(* Logix 5000 AddOnInstructionDefinition export BMC_AOI_PROC_BNI00HM; software revision 20.04 *)

TYPE BMC_UDT_PROC_BNI00HM_Outputs_4277US :   // BNI EIP-508-005-Z015-013Output Map
STRUCT
   Data : INT;
   Restart : INT;
END_STRUCT
END_TYPE

TYPE BMC_UDT_PROC_BNI00HM_Config_4277US :   // BNI EIP-508-005-Z015-013Configuration Map
STRUCT
   Port_1_Function : SINT;   // Sets Port 1 Function 00d=0x00=Standrd I/O 01d=0x01=IO-Link Mod 02d=0x02=Fallback Md
   Port_2_Function : SINT;   // Sets Port 2 Function 00d=0x00=Standrd I/O 01d=0x01=IO-Link Mod 02d=0x02=Fallback Md
   Port_3_Function : SINT;   // Sets Port 3 Function 00d=0x00=Standrd I/O 01d=0x01=IO-Link Mod 02d=0x02=Fallback Md
   Port_4_Function : SINT;   // Sets Port 4 Function 00d=0x00=Standrd I/O 01d=0x01=IO-Link Mod 02d=0x02=Fallback Md
   Port_5_Function : SINT;   // Sets Port 5 Function 00d=0x00=Standrd I/O 01d=0x01=IO-Link Mod 02d=0x02=Fallback Md
   Port_6_Function : SINT;   // Sets Port 6 Function 00d=0x00=Standrd I/O 01d=0x01=IO-Link Mod 02d=0x02=Fallback Md
   Port_7_Function : SINT;   // Sets Port 7 Function 00d=0x00=Standrd I/O 01d=0x01=IO-Link Mod 02d=0x02=Fallback Md
   Port_8_Function : SINT;   // Sets Port 8 Function 00d=0x00=Standrd I/O 01d=0x01=IO-Link Mod 02d=0x02=Fallback Md
   Port_1_Cycle_Time : SINT;   // This SINT is a composite value. Bits 0-5 store Cycle Time Bit 6-7 store Time Base
   Port_1_Validation_Type : SINT;   // Port 1 Validation 00d=0x00=No Validtn 01d=0x01=Compatible [VID + DID]
   Port_1_Vendor_ID_1 : SINT;   // Vendor ID (Hi Byte) of device connected to Port 1 Balluff VID = 378
   Port_1_Vendor_ID_2 : SINT;   // Vendor ID (Lo Byte)
   Port_1_Device_ID_1 : SINT;   // Device ID (Hi Byte) of device connected to Port 1
   Port_1_Device_ID_2 : SINT;   // Device ID (Mid Byte)
   Port_1_Device_ID_3 : SINT;   // Device ID (Low Byte)
   Enable_Upload_Port_1 : BOOL;
   Enable_Download_Port_1 : BOOL;
   Clear_Parameter_Server_Port_1 : BOOL;
   Enable_Parameter_Server_Port_1 : BOOL;
   Port_2_Cycle_Time : SINT;   // This SINT is a composite value. Bits 0-5 store Cycle Time Bit 6-7 store Time Base
   Port_2_Validation_Type : SINT;   // Port 2 Validation 00d=0x00=No Validtn 01d=0x01=Compatible [VID + DID]
   Port_2_Vendor_ID_1 : SINT;   // Vendor ID (Hi Byte) of device connected to Port 2 Balluff VID = 378
   Port_2_Vendor_ID_2 : SINT;   // Vendor ID (Lo Byte)
   Port_2_Device_ID_1 : SINT;   // Device ID (Hi Byte) of device connected to Port 2
   Port_2_Device_ID_2 : SINT;   // Device ID (Mid Byte)
   Port_2_Device_ID_3 : SINT;   // Device ID (Low Byte)
   Enable_Upload_Port_2 : BOOL;
   Enable_Download_Port_2 : BOOL;
   Clear_Parameter_Server_Port_2 : BOOL;
   Enable_Parameter_Server_Port_2 : BOOL;
   Port_3_Cycle_Time : SINT;   // This SINT is a composite value. Bits 0-5 store Cycle Time Bit 6-7 store Time Base
   Port_3_Validation_Type : SINT;   // Port 3 Validation 00d=0x00=No Validtn 01d=0x01=Compatible [VID + DID]
   Port_3_Vendor_ID_1 : SINT;   // Vendor ID (Hi Byte) of device connected to Port 3 Balluff VID = 378
   Port_3_Vendor_ID_2 : SINT;   // Vendor ID (Lo Byte)
   Port_3_Device_ID_1 : SINT;   // Device ID (Hi Byte) of device connected to Port 3
   Port_3_Device_ID_2 : SINT;   // Device ID (Mid Byte)
   Port_3_Device_ID_3 : SINT;   // Device ID (Low Byte)
   Enable_Upload_Port_3 : BOOL;
   Enable_Download_Port_3 : BOOL;
   Clear_Parameter_Server_Port_3 : BOOL;
   Enable_Parameter_Server_Port_3 : BOOL;
   Port_4_Cycle_Time : SINT;   // This SINT is a composite value. Bits 0-5 store Cycle Time Bit 6-7 store Time Base
   Port_4_Validation_Type : SINT;   // Port 4 Validation 00d=0x00=No Validtn 01d=0x01=Compatible [VID + DID]
   Port_4_Vendor_ID_1 : SINT;   // Vendor ID (Hi Byte) of device connected to Port 4 Balluff VID = 378
   Port_4_Vendor_ID_2 : SINT;   // Vendor ID (Lo Byte)
   Port_4_Device_ID_1 : SINT;   // Device ID (Hi Byte) of device connected to Port 4
   Port_4_Device_ID_2 : SINT;   // Device ID (Mid Byte)
   Port_4_Device_ID_3 : SINT;   // Device ID (Low Byte)
   Enable_Upload_Port_4 : BOOL;
   Enable_Download_Port_4 : BOOL;
   Clear_Parameter_Server_Port_4 : BOOL;
   Enable_Parameter_Server_Port_4 : BOOL;
   Port_5_Cycle_Time : SINT;   // This SINT is a composite value. Bits 0-5 store Cycle Time Bit 6-7 store Time Base
   Port_5_Validation_Type : SINT;   // Port 5 Validation 00d=0x00=No Validtn 01d=0x01=Compatible [VID + DID]
   Port_5_Vendor_ID_1 : SINT;   // Vendor ID (Hi Byte) of device connected to Port 5 Balluff VID = 378
   Port_5_Vendor_ID_2 : SINT;   // Vendor ID (Lo Byte)
   Port_5_Device_ID_1 : SINT;   // Device ID (Hi Byte) of device connected to Port 5
   Port_5_Device_ID_2 : SINT;   // Device ID (Mid Byte)
   Port_5_Device_ID_3 : SINT;   // Device ID (Low Byte)
   Enable_Upload_Port_5 : BOOL;
   Enable_Download_Port_5 : BOOL;
   Clear_Parameter_Server_Port_5 : BOOL;
   Enable_Parameter_Server_Port_5 : BOOL;
   Port_6_Cycle_Time : SINT;   // This SINT is a composite value. Bits 0-5 store Cycle Time Bit 6-7 store Time Base
   Port_6_Validation_Type : SINT;   // Port 6 Validation 00d=0x00=No Validtn 01d=0x01=Compatible [VID + DID]
   Port_6_Vendor_ID_1 : SINT;   // Vendor ID (Hi Byte) of device connected to Port 6 Balluff VID = 378
   Port_6_Vendor_ID_2 : SINT;   // Vendor ID (Lo Byte)
   Port_6_Device_ID_1 : SINT;   // Device ID (Hi Byte) of device connected to Port 6
   Port_6_Device_ID_2 : SINT;   // Device ID (Mid Byte)
   Port_6_Device_ID_3 : SINT;   // Device ID (Low Byte)
   Enable_Upload_Port_6 : BOOL;
   Enable_Download_Port_6 : BOOL;
   Clear_Parameter_Server_Port_6 : BOOL;
   Enable_Parameter_Server_Port_6 : BOOL;
   Port_7_Cycle_Time : SINT;   // This SINT is a composite value. Bits 0-5 store Cycle Time Bit 6-7 store Time Base
   Port_7_Validation_Type : SINT;   // Port 7 Validation 00d=0x00=No Validtn 01d=0x01=Compatible [VID + DID]
   Port_7_Vendor_ID_1 : SINT;   // Vendor ID (Hi Byte) of device connected to Port 7 Balluff VID = 378
   Port_7_Vendor_ID_2 : SINT;   // Vendor ID (Lo Byte)
   Port_7_Device_ID_1 : SINT;   // Device ID (Hi Byte) of device connected to Port 7
   Port_7_Device_ID_2 : SINT;   // Device ID (Mid Byte)
   Port_7_Device_ID_3 : SINT;   // Device ID (Low Byte)
   Enable_Upload_Port_7 : BOOL;
   Enable_Download_Port_7 : BOOL;
   Clear_Parameter_Server_Port_7 : BOOL;
   Enable_Parameter_Server_Port_7 : BOOL;
   Port_8_Cycle_Time : SINT;   // This SINT is a composite value. Bits 0-5 store Cycle Time Bit 6-7 store Time Base
   Port_8_Validation_Type : SINT;   // Port 8 Validation 00d=0x00=No Validtn 01d=0x01=Compatible [VID + DID]
   Port_8_Vendor_ID_1 : SINT;   // Vendor ID (Hi Byte) of device connected to Port 8 Balluff VID = 378
   Port_8_Vendor_ID_2 : SINT;   // Vendor ID (Lo Byte)
   Port_8_Device_ID_1 : SINT;   // Device ID (Hi Byte) of device connected to Port 8
   Port_8_Device_ID_2 : SINT;   // Device ID (Mid Byte)
   Port_8_Device_ID_3 : SINT;   // Device ID (Low Byte)
   Enable_Upload_Port_8 : BOOL;
   Enable_Download_Port_8 : BOOL;
   Clear_Parameter_Server_Port_8 : BOOL;
   Enable_Parameter_Server_Port_8 : BOOL;
END_STRUCT
END_TYPE

TYPE BMC_UDT_PROC_BNI00HM_Data_4277US :   // BNI EIP-508-005-Z015-013IO Map
STRUCT
   I : BMC_UDT_PROC_BNI00HM_Inputs_4277US;
   O : BMC_UDT_PROC_BNI00HM_Outputs_4277US;
   C : BMC_UDT_PROC_BNI00HM_Config_4277US;
END_STRUCT
END_TYPE

TYPE BMC_UDT_PROC_BNI00HM_Inputs_4277US :   // BNI EIP-508-005-Z015-013 Input Map
STRUCT
   Data : INT;
   Short_Circuit : INT;
   Overload : INT;
   UA_Fault : BOOL;
   US_Fault : BOOL;
   Port_1_IO_Link_Status : BOOL;
   Port_1_Device_Connected : BOOL;
   Port_1_Validation_Failed : BOOL;
   Port_2_IO_Link_Status : BOOL;
   Port_2_Device_Connected : BOOL;
   Port_2_Validation_Failed : BOOL;
   Port_3_IO_Link_Status : BOOL;
   Port_3_Device_Connected : BOOL;
   Port_3_Validation_Failed : BOOL;
   Port_4_IO_Link_Status : BOOL;
   Port_4_Device_Connected : BOOL;
   Port_4_Validation_Failed : BOOL;
   Port_5_IO_Link_Status : BOOL;
   Port_5_Device_Connected : BOOL;
   Port_5_Validation_Failed : BOOL;
   Port_6_IO_Link_Status : BOOL;
   Port_6_Device_Connected : BOOL;
   Port_6_Validation_Failed : BOOL;
   Port_7_IO_Link_Status : BOOL;
   Port_7_Device_Connected : BOOL;
   Port_7_Validation_Failed : BOOL;
   Port_8_IO_Link_Status : BOOL;
   Port_8_Device_Connected : BOOL;
   Port_8_Validation_Failed : BOOL;
END_STRUCT
END_TYPE

TYPE IO_Link_Port_Data :
STRUCT
   Inputs : SINT[48];
   Outputs : SINT[48];
END_STRUCT
END_TYPE

ADD_ON_INSTRUCTION BMC_AOI_PROC_BNI00HM   (* revision 4.0, vendor Balluff Inc *)
// BNI EIP-508-005-Z015-013
// HW9 EIP IOL Master
// Revision note:
// Initial Release:
// xx1323US V4.0
// Initial Revision:
// xx4722US  V3.0
VAR_IN_OUT
   BNI_EIP_508_Raw_Input_Data : SINT[392]; {required}
        [0].0   // Input Port 0 Pin 4
        [0].1   // Input Port 0 Pin 2
        [0].2   // Input Port 1 Pin 4
        [0].3   // Input Port 1 Pin 2
        [0].4   // Input Port 2 Pin 4
        [0].5   // Input Port 2 Pin 2
        [0].6   // Input Port 3 Pin 4
        [0].7   // Input Port 3 Pin 2
        [1].0   // Input Port 4 Pin 4
        [1].1   // Input Port 4 Pin 2
        [1].2   // Input Port 5 Pin 4
        [1].3   // Input Port 5 Pin 2
        [1].4   // Input Port 6 Pin 4
        [1].5   // Input Port 6 Pin 2
        [1].6   // Input Port 7 Pin 4
        [1].7   // Input Port 7 Pin 2
        [2].0   // Port 0 Pin 4 Short Circuit
        [2].1   // Port 0 Pin 2 Short Circuit
        [2].2   // Port 1 Pin 4 Short Circuit
        [2].3   // Port 1 Pin 2 Short Circuit
        [2].4   // Port 2 Pin 4 Short Circuit
        [2].5   // Port 2 Pin 2 Short Circuit
        [2].6   // Port 3 Pin 4 Short Circuit
        [2].7   // Port 3 Pin 2 Short Circuit
        [3].0   // Port 4 Pin 4 Short Circuit
        [3].1   // Port 4 Pin 2 Short Circuit
        [3].2   // Port 5 Pin 4 Short Circuit
        [3].3   // Port 5 Pin 2 Short Circuit
        [3].4   // Port 6 Pin 4 Short Circuit
        [3].5   // Port 6 Pin 2 Short Circuit
        [3].6   // Port 7 Pin 4 Short Circuit
        [3].7   // Port 7 Pin 2 Short Circuit
        [4].0   // Port 0 Pin 4 Output Overload Status
        [4].1   // Port 0 Pin 2 Output Overload Status
        [4].2   // Port 1 Pin 4 Output Overload Status
        [4].3   // Port 1 Pin 2 Output Overload Status
        [4].4   // Port 2 Pin 4 Output Overload Status
        [4].5   // Port 2 Pin 2 Output Overload Status
        [4].6   // Port 3 Pin 4 Output Overload Status
        [4].7   // Port 3 Pin 2 Output Overload Status
        [5].0   // Port 4 Pin 4 Output Overload Status
        [5].1   // Port 4 Pin 2 Output Overload Status
        [5].2   // Port 5 Pin 4 Output Overload Status
        [5].3   // Port 5 Pin 2 Output Overload Status
        [5].4   // Port 6 Pin 4 Output Overload Status
        [5].5   // Port 6 Pin 2 Output Overload Status
        [5].6   // Port 7 Pin 4 Output Overload Status
        [5].7   // Port 7 Pin 2 Output Overload Status
        [6].0   // Output Power from Aux Power cable Under Voltage
        [6].1   // Module Power from IO-Link Communication Cable Under Voltage
        [6].2   // Not used
        [6].3   // Not used
        [6].4   // Not used
        [6].5   // Not used
        [6].6   // Not used
        [6].7   // Not used
        [7]   // Port 1 Input Byte 0
        [8]   // Port 1 Input Byte 1
        [9]   // Port 1 Input Byte 2
        [10]   // Port 1 Input Byte 3
        [11]   // Port 1 Input Byte 4
        [32].0   // Port 1 EP bit Event Present
        [32].1   // Reserved
        [32].2   // Reserved
        [32].3   // Reserved
        [32].4   // Reserved
        [32].5   // Port 1 VF bit Validation Failed
        [32].6   // Port 1 DC bit Device Connected
        [32].7   // Port 1 IOL bit Port in IO-Link Mode
        [33].0   // Reserved
        [33].1   // Reserved
        [33].2   // Reserved
        [33].3   // Reserved
        [33].4   // Reserved
        [33].5   // Reserved
        [33].6   // Reserved
        [33].7   // Reserved
        [34]   // Port 1 Vendor ID Number Byte 1 (High byte)
        [35]   // Port 1 Vendor ID Number Byte 2 (Middle byte)
        [36]   // Port 1 Vendor ID Number Byte 3 (Low byte)
        [37]   // Port 1 Device ID Number Byte 1 (High byte)
        [38]   // Port 1 Device ID Number Byte 2 (Middle byte)
        [39]   // Port 1 Device ID Number Byte 3 (Low byte)
        [40].0   // Port 1 In I/O Link Mode
        [40].1   // Port 1 I/O Link Device Connected
        [41].0   // Port 1 I/O Link Device Configuration Mismatch
        [52]   // Port 1 Input Byte 46
        [53]   // Port 1 Input Byte 47
        [54]   // Port 1 Input Byte 48
        [55]   // Port 2 Input Byte 0
        [56]   // Port 2 Input Byte 1
        [57]   // Port 2 Input Byte 2
        [58]   // Port 2 Input Byte 3
        [59]   // Port 2 Input Byte 4
        [88].0   // Port 2 In I/O Link Mode
        [88].1   // Port 2 I/O Link Device Connected
        [89].0   // Port 2 I/O Link Device Configuration Mismatch
        [100]   // Port 2 Input Byte 46
        [101]   // Port 2 Input Byte 47
        [102]   // Port 2 Input Byte 48
        [103]   // Port 3 Input Byte 0
        [104]   // Port 3 Input Byte 1
        [105]   // Port 3 Input Byte 2
        [106]   // Port 3 Input Byte 3
        [107]   // Port 3 Input Byte 4
        [136].0   // Port 3 In I/O Link Mode
        [136].1   // Port 3 I/O Link Device Connected
        [137].0   // Port 3 I/O Link Device Configuration Mismatch
        [148]   // Port 3 Input Byte 46
        [149]   // Port 3 Input Byte 47
        [150]   // Port 3 Input Byte 48
        [151]   // Port 4 Input Byte 0
        [152]   // Port 4 Input Byte 1
        [153]   // Port 4 Input Byte 2
        [154]   // Port 4 Input Byte 3
        [184].0   // Port 4 In I/O Link Mode
        [184].1   // Port 4 I/O Link Device Connected
        [185].0   // Port 4 I/O Link Device Configuration Mismatch
        [196]   // Port 4 Input Byte 46
        [197]   // Port 4 Input Byte 47
        [198]   // Port 4 Input Byte 48
   BNI_EIP_508_Raw_Output_Data : SINT[262]; {required}
        [0].0   // Output Port 0 Pin 4
        [0].1   // Output Port 0 Pin 2
        [0].2   // Output Port 1 Pin 4
        [0].3   // Output Port 1 Pin 2
        [0].4   // Output Port 2 Pin 4
        [0].5   // Output Port 2 Pin 2
        [0].6   // Output Port 3 Pin 4
        [0].7   // Output Port 3 Pin 2
        [1].0   // Output Port 4 Pin 4
        [1].1   // Output Port 4 Pin 2
        [1].2   // Output Port 5 Pin 4
        [1].3   // Output Port 5 Pin 2
        [1].4   // Output Port 6 Pin 4
        [1].5   // Output Port 6 Pin 2
        [1].6   // Output Port 7 Pin 4
        [1].7   // Output Port 7 Pin 2
        [2].0   // Port 0 Pin 4 Output Restart
        [2].1   // Port 0 Pin 2 Output Restart
        [2].2   // Port 1 Pin 4 Output Restart
        [2].3   // Port 1 Pin 2 Output Restart
        [2].4   // Port 2 Pin 4 Output Restart
        [2].5   // Port 2 Pin 2 Output Restart
        [2].6   // Port 3 Pin 4 Output Restart
        [2].7   // Port 3 Pin 2 Output Restart
        [3].0   // Port 4 Pin 4 Output Restart
        [3].1   // Port 4 Pin 2 Output Restart
        [3].2   // Port 5 Pin 4 Output Restart
        [3].3   // Port 5 Pin 2 Output Restart
        [3].4   // Port 6 Pin 4 Output Restart
        [3].5   // Port 6 Pin 2 Output Restart
        [3].6   // Port 7 Pin 4 Output Restart
        [3].7   // Port 7 Pin 2 Output Restart
        [4].0   // Red LED Display Output
        [4].1   // Green LED Display Output
        [4].2   // Lock Display Output
        [5]   // Port 1 Output Data Byte 0
        [6]   // Port 1 Output Data Byte 1
        [7]   // Port 1 Output Data Byte 2
        [8]   // Port 1 Output Data Byte 3
        [9]   // Port 1 Output Data Byte 4
        [10]   // Port 1 Output Data Byte 5
        [11]   // Port 1 Output Data Byte 6
        [12]   // Port 1 Output Data Byte 7
        [13]   // Port 1 Output Data Byte 8
        [14]   // Port 1 Output Data Byte 9
        [15]   // Port 1 Output Data Byte 10
        [16]   // Port 1 Output Data Byte 11
        [17]   // Port 1 Output Data Byte 12
        [18]   // Port 1 Output Data Byte 13
        [19]   // Port 1 Output Data Byte 14
        [20]   // Port 1 Output Data Byte 15
        [21]   // Port 1 Output Data Byte 16
        [22]   // Port 1 Output Data Byte 17
        [23]   // Port 1 Output Data Byte 18
        [24]   // Port 1 Output Data Byte 19
        [25]   // Port 1 Output Data Byte 20
        [26]   // Port 1 Output Data Byte 21
        [27]   // Port 1 Output Data Byte 22
        [28]   // Port 1 Output Data Byte 23
        [29]   // Port 1 Output Data Byte 24
        [30]   // Port 1 Output Data Byte 25
        [31]   // Port 1 Output Data Byte 26
        [32]   // Port 1 Output Data Byte 27
        [33]   // Port 1 Output Data Byte 28
        [34]   // Port 1 Output Data Byte 29
        [35]   // Port 1 Output Data Byte 30
        [36]   // Port 1 Output Data Byte 31
        [37]   // Port 2 Output Data Byte 0
        [38]   // Port 2 Output Data Byte 1
        [69]   // Port 3 Output Data Byte 0
        [70]   // Port 3 Output Data Byte 1
        [101]   // Port 4 Output Data Byte 0
        [102]   // Port 4 Output Data Byte 1
   BNI_EIP_508_Raw_Config_Data : SINT[194]; {required}
        [0]   // Port 1(Bits 0_1) Port 2 (Bits 2_3) Port 3 (Bits 4_5) Port 4 (Bits 6_7) Function 00d=0x00=Standrd I/O 01d=0x01=IO-Link Mod
        [1]   // Port 5 (Bits 0_1) Port 6 (Bits 2_3) Port 7 (Bits 4_5) Port 8 (Bits 6_7) Function Function 00d=0x00=Standrd I/O 01d=0x01=IO-Link Mod
        [2].0   // Parameter Data Conflict
        [2].1   // Enable Parameter Upload
        [2].2   // Enable Parameter Download
        [2].7   // Enable Parameter Server
        [3]   // RESERVED
        [4]   // Port 1 IO-Link Cycle Time Time (Bytes 5-0) Base (Bytes 7-6)
        [5]   // Port 1 Vendor ID Number Byte 1 High Byte
        [6]   // Port 1 Vendor ID Number Byte 2 Low Byte
        [7]   // Port 1 Device ID Number Byte 1 High Byte
        [8]   // Port 1 Device ID Number Byte 2 Middle Byte
        [9]   // Port 1 Device ID Number Byte 3 Low Byte
        [10]   // Port 2 IO-Link Cycle Time Time (Bytes 5-0) Base (Bytes 7-6)
        [11]   // Port 2 Vendor ID Number Byte 1 High Byte
        [12]   // Port 2 Vendor ID Number Byte 2 Low Byte
        [13]   // Port 2 Device ID Number Byte 1 High Byte
        [14]   // Port 2 Device ID Number Byte 2 Middle Byte
        [15]   // Port 2 Device ID Number Byte 3 Low Byte
        [16]   // Port 3 IO-Link Cycle Time Time (Bytes 5-0) Base (Bytes 7-6)
        [17]   // Port 3 Vendor ID Number Byte 1 High Byte
        [18]   // Port 3 Vendor ID Number Byte 2 Low Byte
        [19]   // Port 3 Device ID Number Byte 1 High Byte
        [20]   // Port 3 Device ID Number Byte 2 Middle Byte
        [21]   // Port 3 Device ID Number Byte 3 Low Byte
        [22]   // Port 4 IO-Link Cycle Time Time (Bytes 5-0) Base (Bytes 7-6)
        [23]   // Port 4 Vendor ID Number Byte 1 High Byte
        [24]   // Port 4 Vendor ID Number Byte 2 Low Byte
        [25]   // Port 1 Enable
        [25].1   // Port 1 Enable Upload Parameters
        [25].2   // Port 1 Enable Download Parameters
        [25].7   // Port 1 Enable Parameters Server
        [26]   // Port 4 Device ID Number Byte 2 Middle Byte
        [27]   // Port 4 Device ID Number Byte 3 Low Byte
        [49].1   // Port 2 Enable Upload Parameters
        [49].2   // Port 2 Enable Download Parameters
        [49].7   // Port 2 Enable Parameters Server
        [73].1   // Port 3 Enable Upload Parameters
        [73].2   // Port 3 Enable Download Parameters
        [73].7   // Port 3 Enable Parameters Server
        [97].1   // Port 4 Enable Upload Parameters
        [97].2   // Port 4 Enable Download Parameters
        [97].7   // Port 4 Enable Parameters Server
   BNI_EIP_508_Port_1_Data : IO_Link_Port_Data; {required}
        .INPUTS[0]   // Port 1 Input Data
   BNI_EIP_508_Port_2_Data : IO_Link_Port_Data; {required}
        .INPUTS[0]   // Port 2 Input Data
   BNI_EIP_508_Port_3_Data : IO_Link_Port_Data; {required}
        .INPUTS[0]   // Port 3 Input Data
   BNI_EIP_508_Port_4_Data : IO_Link_Port_Data; {required}
        .INPUTS[0]   // Port 4 Input Data
   BNI_EIP_508_Port_5_Data : IO_Link_Port_Data; {required}
   BNI_EIP_508_Port_6_Data : IO_Link_Port_Data; {required}
   BNI_EIP_508_Port_7_Data : IO_Link_Port_Data; {required}
   BNI_EIP_508_Port_8_Data : IO_Link_Port_Data; {required}
   Mapped_BNI_EIP_508_Data : BMC_UDT_PROC_BNI00HM_Data_4277US; {required}
        .I.DATA.0   // Input Port 0 Pin 4
        .I.DATA.1   // Input Port 0 Pin 2
        .I.DATA.2   // Input Port 1 Pin 4
        .I.DATA.3   // Input Port 1 Pin 2
        .I.DATA.4   // Input Port 2 Pin 4
        .I.DATA.5   // Input Port 2 Pin 2
        .I.DATA.6   // Input Port 3 Pin 4
        .I.DATA.7   // Input Port 3 Pin 2
        .I.DATA.8   // Input Port 4 Pin 4
        .I.DATA.9   // Input Port 4 Pin 2
        .I.DATA.10   // Input Port 5 Pin 4
        .I.DATA.11   // Input Port 5 Pin 2
        .I.DATA.12   // Input Port 6 Pin 4
        .I.DATA.13   // Input Port 6 Pin 2
        .I.DATA.14   // Input Port 7 Pin 4
        .I.DATA.15   // Input Port 7 Pin 2
        .I.SHORT_CIRCUIT.0   // Port 0 Pin 4 Short Circuit
        .I.SHORT_CIRCUIT.1   // Port 0 Pin 2 Short Circuit
        .I.SHORT_CIRCUIT.2   // Port 1 Pin 4 Short Circuit
        .I.SHORT_CIRCUIT.3   // Port 1 Pin 2 Short Circuit
        .I.SHORT_CIRCUIT.4   // Port 2 Pin 4 Short Circuit
        .I.SHORT_CIRCUIT.5   // Port 2 Pin 2 Short Circuit
        .I.SHORT_CIRCUIT.6   // Port 3 Pin 4 Short Circuit
        .I.SHORT_CIRCUIT.7   // Port 3 Pin 2 Short Circuit
        .I.SHORT_CIRCUIT.8   // Port 4 Pin 4 Short Circuit
        .I.SHORT_CIRCUIT.9   // Port 4 Pin 2 Short Circuit
        .I.SHORT_CIRCUIT.10   // Port 5 Pin 4 Short Circuit
        .I.SHORT_CIRCUIT.11   // Port 5 Pin 2 Short Circuit
        .I.SHORT_CIRCUIT.12   // Port 6 Pin 4 Short Circuit
        .I.SHORT_CIRCUIT.13   // Port 6 Pin 2 Short Circuit
        .I.SHORT_CIRCUIT.14   // Port 7 Pin 4 Short Circuit
        .I.SHORT_CIRCUIT.15   // Port 7 Pin 2 Short Circuit
        .I.OVERLOAD.0   // Port 0 Pin 4 Output Overload Status
        .I.OVERLOAD.1   // Port 0 Pin 2 Output Overload Status
        .I.OVERLOAD.2   // Port 1 Pin 4 Output Overload Status
        .I.OVERLOAD.3   // Port 1 Pin 2 Output Overload Status
        .I.OVERLOAD.4   // Port 2 Pin 4 Output Overload Status
        .I.OVERLOAD.5   // Port 2 Pin 2 Output Overload Status
        .I.OVERLOAD.6   // Port 3 Pin 4 Output Overload Status
        .I.OVERLOAD.7   // Port 3 Pin 2 Output Overload Status
        .I.OVERLOAD.8   // Port 4 Pin 4 Output Overload Status
        .I.OVERLOAD.9   // Port 4 Pin 2 Output Overload Status
        .I.OVERLOAD.10   // Port 5 Pin 4 Output Overload Status
        .I.OVERLOAD.11   // Port 5 Pin 2 Output Overload Status
        .I.OVERLOAD.12   // Port 6 Pin 4 Output Overload Status
        .I.OVERLOAD.13   // Port 6 Pin 2 Output Overload Status
        .I.OVERLOAD.14   // Port 7 Pin 4 Output Overload Status
        .I.OVERLOAD.15   // Port 7 Pin 2 Output Overload Status
        .I.UA_FAULT   // Output Power from Aux Power cable Under Voltage
        .I.US_FAULT   // Module Power from IO-Link Communication Cable Under Voltage
        .I.PORT_1_IO_LINK_STATUS   // Port 1 In I/O Link Mode
        .I.PORT_1_DEVICE_CONNECTED   // Port 1 I/O Link Device Connected
        .I.PORT_1_VALIDATION_FAILED   // Port 1 I/O Link Device Configuration Mismatch
        .I.PORT_2_IO_LINK_STATUS   // Port 2 In I/O Link Mode
        .I.PORT_2_DEVICE_CONNECTED   // Port 2 I/O Link Device Connected
        .I.PORT_2_VALIDATION_FAILED   // Port 2 I/O Link Device Configuration Mismatch
        .I.PORT_3_IO_LINK_STATUS   // Port 3 In I/O Link Mode
        .I.PORT_3_DEVICE_CONNECTED   // Port 3 I/O Link Device Connected
        .I.PORT_3_VALIDATION_FAILED   // Port 3 I/O Link Device Configuration Mismatch
        .I.PORT_4_IO_LINK_STATUS   // Port 4 In I/O Link Mode
        .I.PORT_4_DEVICE_CONNECTED   // Port 4 I/O Link Device Connected
        .I.PORT_4_VALIDATION_FAILED   // Port 4 I/O Link Device Configuration Mismatch
        .O.DATA.0   // Output Port 0 Pin 4
        .O.DATA.1   // Output Port 0 Pin 2
        .O.DATA.2   // Output Port 1 Pin 4
        .O.DATA.3   // Output Port 1 Pin 2
        .O.DATA.4   // Output Port 2 Pin 4
        .O.DATA.5   // Output Port 2 Pin 2
        .O.DATA.6   // Output Port 3 Pin 4
        .O.DATA.7   // Output Port 3 Pin 2
        .O.DATA.8   // Output Port 4 Pin 4
        .O.DATA.9   // Output Port 4 Pin 2
        .O.DATA.10   // Output Port 5 Pin 4
        .O.DATA.11   // Output Port 5 Pin 2
        .O.DATA.12   // Output Port 6 Pin 4
        .O.DATA.13   // Output Port 6 Pin 2
        .O.DATA.14   // Output Port 7 Pin 4
        .O.DATA.15   // Output Port 7 Pin 2
        .O.DISPLAY_GREEN   // Green LED On
        .O.DISPLAY_LOCK   // Display Lock PLC Lock
        .O.DISPLAY_RED   // Red LED On
        .O.RESTART.0   // Port 0 Pin 4 Output Restart
        .O.RESTART.1   // Port 0 Pin 2 Output Restart
        .O.RESTART.2   // Port 1 Pin 4 Output Restart
        .O.RESTART.3   // Port 1 Pin 2 Output Restart
        .O.RESTART.4   // Port 2 Pin 4 Output Restart
        .O.RESTART.5   // Port 2 Pin 2 Output Restart
        .O.RESTART.6   // Port 3 Pin 4 Output Restart
        .O.RESTART.7   // Port 3 Pin 2 Output Restart
        .O.RESTART.8   // Port 4 Pin 4 Output Restart
        .O.RESTART.9   // Port 4 Pin 2 Output Restart
        .O.RESTART.10   // Port 5 Pin 4 Output Restart
        .O.RESTART.11   // Port 5 Pin 2 Output Restart
        .O.RESTART.12   // Port 6 Pin 4 Output Restart
        .O.RESTART.13   // Port 6 Pin 2 Output Restart
        .O.RESTART.14   // Port 7 Pin 4 Output Restart
        .O.RESTART.15   // Port 7 Pin 2 Output Restart
END_VAR
VAR
   Clear_Parameter_Server_Port_1 : BOOL; {access None}
END_VAR

ROUTINE Logic   (* ladder *)
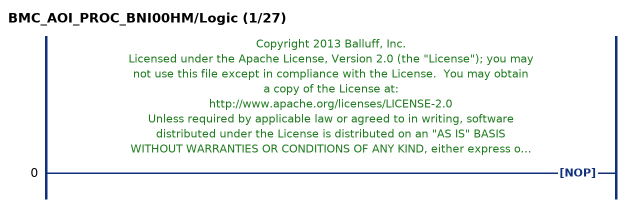
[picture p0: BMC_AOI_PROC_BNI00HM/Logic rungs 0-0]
   // Copyright 2013 Balluff, Inc.
   // Licensed under the Apache License, Version 2.0 (the "License"); you may
   // not use this file except in compliance with the License.  You may obtain
   // a copy of the License at:
   // http://www.apache.org/licenses/LICENSE-2.0
   // Unless required by applicable law or agreed to in writing, software
   // distributed under the License is distributed on an "AS IS" BASIS
   // WITHOUT WARRANTIES OR CONDITIONS OF ANY KIND, either express or
   // implied.  See the License for the specific language governing
   // permissions and limitations under the License.
   0: NOP();
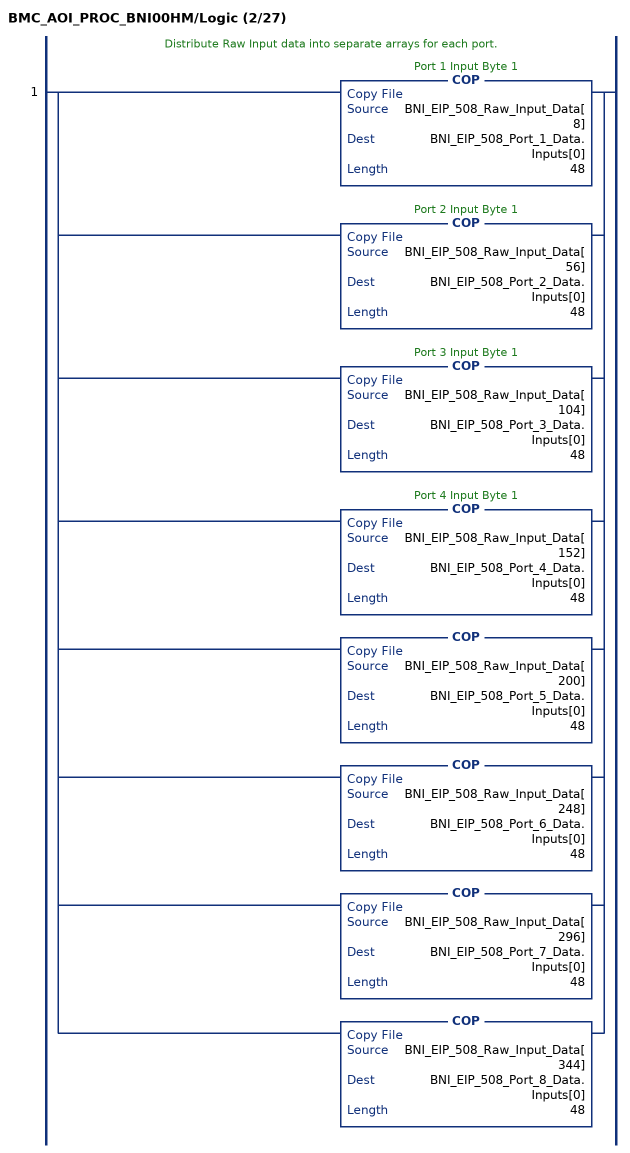
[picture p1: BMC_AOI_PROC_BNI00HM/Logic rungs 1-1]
   // Distribute Raw Input data into separate arrays for each port.
   1: [COP(BNI_EIP_508_Raw_Input_Data[8],BNI_EIP_508_Port_1_Data.Inputs[0],48) ,COP(BNI_EIP_508_Raw_Input_Data[56],BNI_EIP_508_Port_2_Data.Inputs[0],48) ,COP(BNI_EIP_508_Raw_Input_Data[104],BNI_EIP_508_Port_3_Data.Inputs[0],48) ,COP(BNI_EIP_508_Raw_Input_Data[152],BNI_EIP_508_Port_4_Data.Inputs[0],48) ,COP(BNI_EIP_508_Raw_Input_Data[200],BNI_EIP_508_Port_5_Data.Inputs[0],48) ,COP(BNI_EIP_508_Raw_Input_Data[248],BNI_EIP_508_Port_6_Data.Inputs[0],48) ,COP(BNI_EIP_508_Raw_Input_Data[296],BNI_EIP_508_Port_7_Data.Inputs[0],48) ,COP(BNI_EIP_508_Raw_Input_Data[344],BNI_EIP_508_Port_8_Data.Inputs[0],48) ];
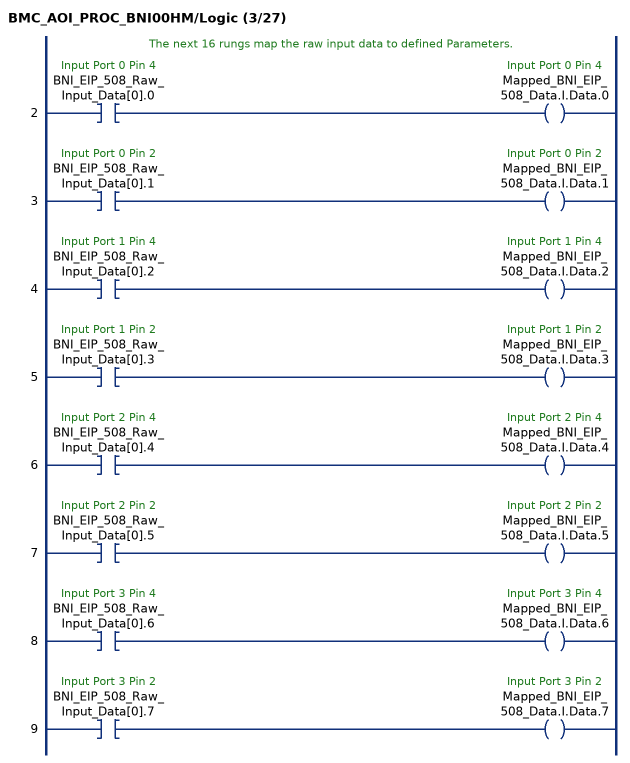
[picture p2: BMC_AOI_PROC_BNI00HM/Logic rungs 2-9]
   // The next 16 rungs map the raw input data to defined Parameters.
   2: XIC(BNI_EIP_508_Raw_Input_Data[0].0)OTE(Mapped_BNI_EIP_508_Data.I.Data.0);
   3: XIC(BNI_EIP_508_Raw_Input_Data[0].1)OTE(Mapped_BNI_EIP_508_Data.I.Data.1);
   4: XIC(BNI_EIP_508_Raw_Input_Data[0].2)OTE(Mapped_BNI_EIP_508_Data.I.Data.2);
   5: XIC(BNI_EIP_508_Raw_Input_Data[0].3)OTE(Mapped_BNI_EIP_508_Data.I.Data.3);
   6: XIC(BNI_EIP_508_Raw_Input_Data[0].4)OTE(Mapped_BNI_EIP_508_Data.I.Data.4);
   7: XIC(BNI_EIP_508_Raw_Input_Data[0].5)OTE(Mapped_BNI_EIP_508_Data.I.Data.5);
   8: XIC(BNI_EIP_508_Raw_Input_Data[0].6)OTE(Mapped_BNI_EIP_508_Data.I.Data.6);
   9: XIC(BNI_EIP_508_Raw_Input_Data[0].7)OTE(Mapped_BNI_EIP_508_Data.I.Data.7);
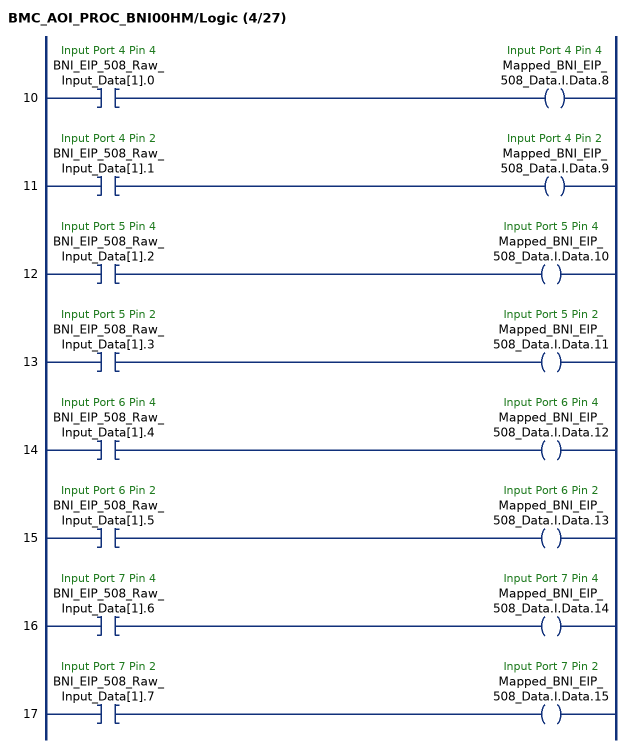
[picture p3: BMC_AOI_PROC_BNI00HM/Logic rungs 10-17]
   10: XIC(BNI_EIP_508_Raw_Input_Data[1].0)OTE(Mapped_BNI_EIP_508_Data.I.Data.8);
   11: XIC(BNI_EIP_508_Raw_Input_Data[1].1)OTE(Mapped_BNI_EIP_508_Data.I.Data.9);
   12: XIC(BNI_EIP_508_Raw_Input_Data[1].2)OTE(Mapped_BNI_EIP_508_Data.I.Data.10);
   13: XIC(BNI_EIP_508_Raw_Input_Data[1].3)OTE(Mapped_BNI_EIP_508_Data.I.Data.11);
   14: XIC(BNI_EIP_508_Raw_Input_Data[1].4)OTE(Mapped_BNI_EIP_508_Data.I.Data.12);
   15: XIC(BNI_EIP_508_Raw_Input_Data[1].5)OTE(Mapped_BNI_EIP_508_Data.I.Data.13);
   16: XIC(BNI_EIP_508_Raw_Input_Data[1].6)OTE(Mapped_BNI_EIP_508_Data.I.Data.14);
   17: XIC(BNI_EIP_508_Raw_Input_Data[1].7)OTE(Mapped_BNI_EIP_508_Data.I.Data.15);
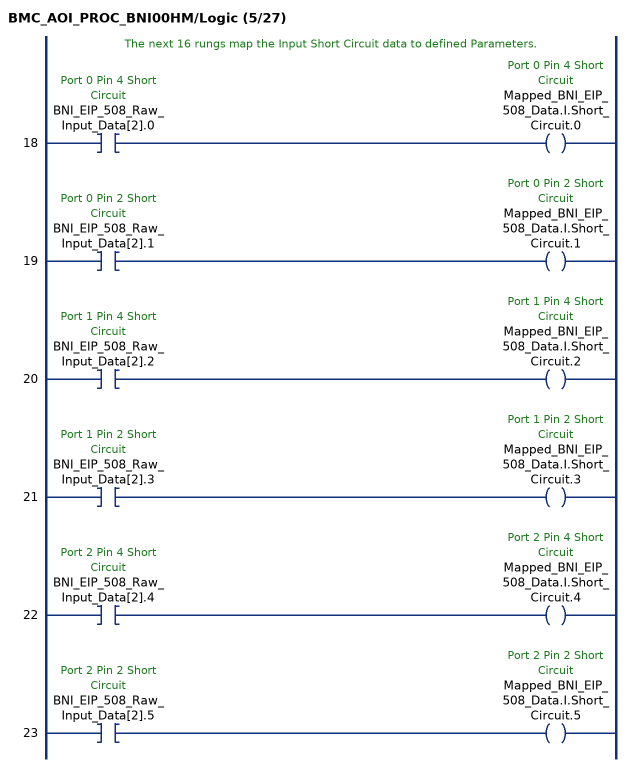
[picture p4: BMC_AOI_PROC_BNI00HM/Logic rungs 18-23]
   // The next 16 rungs map the Input Short Circuit data to defined Parameters.
   18: XIC(BNI_EIP_508_Raw_Input_Data[2].0)OTE(Mapped_BNI_EIP_508_Data.I.Short_Circuit.0);
   19: XIC(BNI_EIP_508_Raw_Input_Data[2].1)OTE(Mapped_BNI_EIP_508_Data.I.Short_Circuit.1);
   20: XIC(BNI_EIP_508_Raw_Input_Data[2].2)OTE(Mapped_BNI_EIP_508_Data.I.Short_Circuit.2);
   21: XIC(BNI_EIP_508_Raw_Input_Data[2].3)OTE(Mapped_BNI_EIP_508_Data.I.Short_Circuit.3);
   22: XIC(BNI_EIP_508_Raw_Input_Data[2].4)OTE(Mapped_BNI_EIP_508_Data.I.Short_Circuit.4);
   23: XIC(BNI_EIP_508_Raw_Input_Data[2].5)OTE(Mapped_BNI_EIP_508_Data.I.Short_Circuit.5);
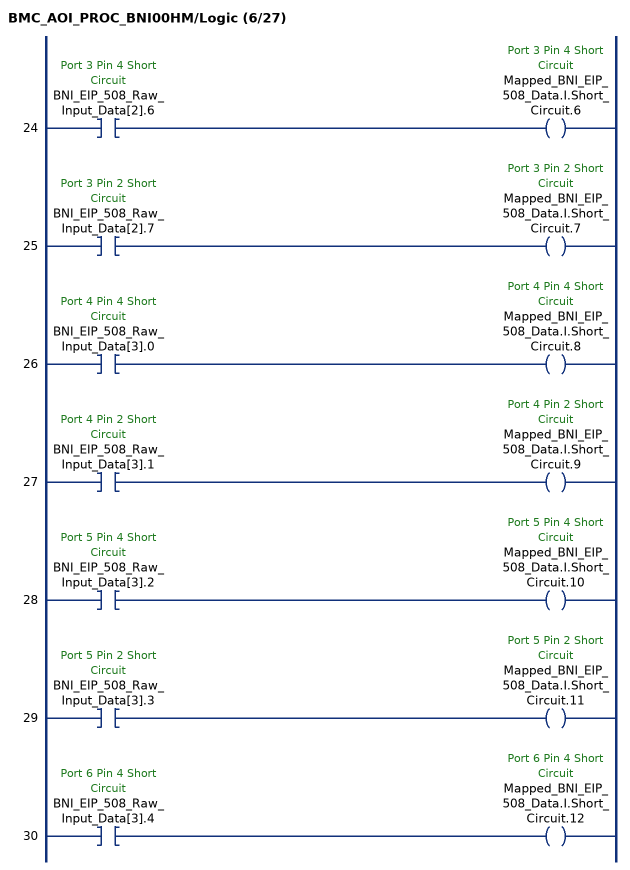
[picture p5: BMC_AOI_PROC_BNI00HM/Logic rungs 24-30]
   24: XIC(BNI_EIP_508_Raw_Input_Data[2].6)OTE(Mapped_BNI_EIP_508_Data.I.Short_Circuit.6);
   25: XIC(BNI_EIP_508_Raw_Input_Data[2].7)OTE(Mapped_BNI_EIP_508_Data.I.Short_Circuit.7);
   26: XIC(BNI_EIP_508_Raw_Input_Data[3].0)OTE(Mapped_BNI_EIP_508_Data.I.Short_Circuit.8);
   27: XIC(BNI_EIP_508_Raw_Input_Data[3].1)OTE(Mapped_BNI_EIP_508_Data.I.Short_Circuit.9);
   28: XIC(BNI_EIP_508_Raw_Input_Data[3].2)OTE(Mapped_BNI_EIP_508_Data.I.Short_Circuit.10);
   29: XIC(BNI_EIP_508_Raw_Input_Data[3].3)OTE(Mapped_BNI_EIP_508_Data.I.Short_Circuit.11);
   30: XIC(BNI_EIP_508_Raw_Input_Data[3].4)OTE(Mapped_BNI_EIP_508_Data.I.Short_Circuit.12);
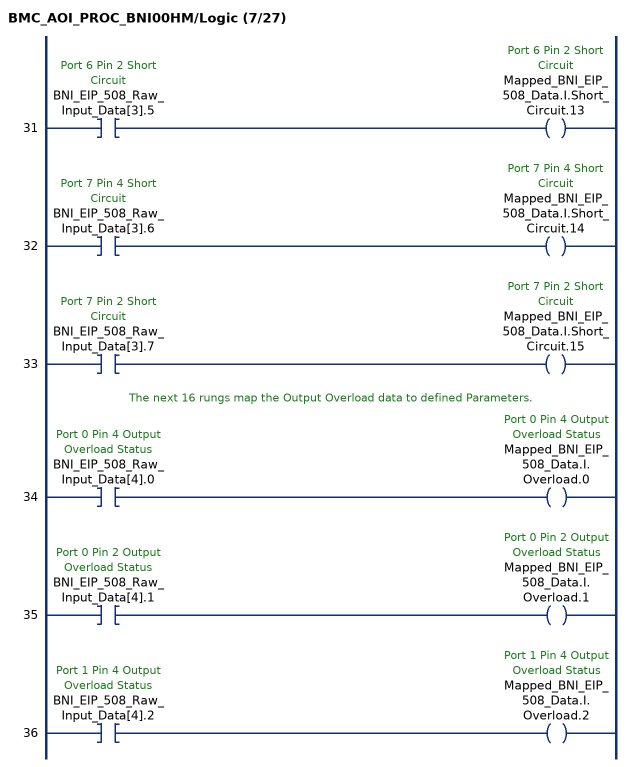
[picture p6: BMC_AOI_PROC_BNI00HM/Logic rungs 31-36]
   31: XIC(BNI_EIP_508_Raw_Input_Data[3].5)OTE(Mapped_BNI_EIP_508_Data.I.Short_Circuit.13);
   32: XIC(BNI_EIP_508_Raw_Input_Data[3].6)OTE(Mapped_BNI_EIP_508_Data.I.Short_Circuit.14);
   33: XIC(BNI_EIP_508_Raw_Input_Data[3].7)OTE(Mapped_BNI_EIP_508_Data.I.Short_Circuit.15);
   // The next 16 rungs map the Output Overload data to defined Parameters.
   34: XIC(BNI_EIP_508_Raw_Input_Data[4].0)OTE(Mapped_BNI_EIP_508_Data.I.Overload.0);
   35: XIC(BNI_EIP_508_Raw_Input_Data[4].1)OTE(Mapped_BNI_EIP_508_Data.I.Overload.1);
   36: XIC(BNI_EIP_508_Raw_Input_Data[4].2)OTE(Mapped_BNI_EIP_508_Data.I.Overload.2);
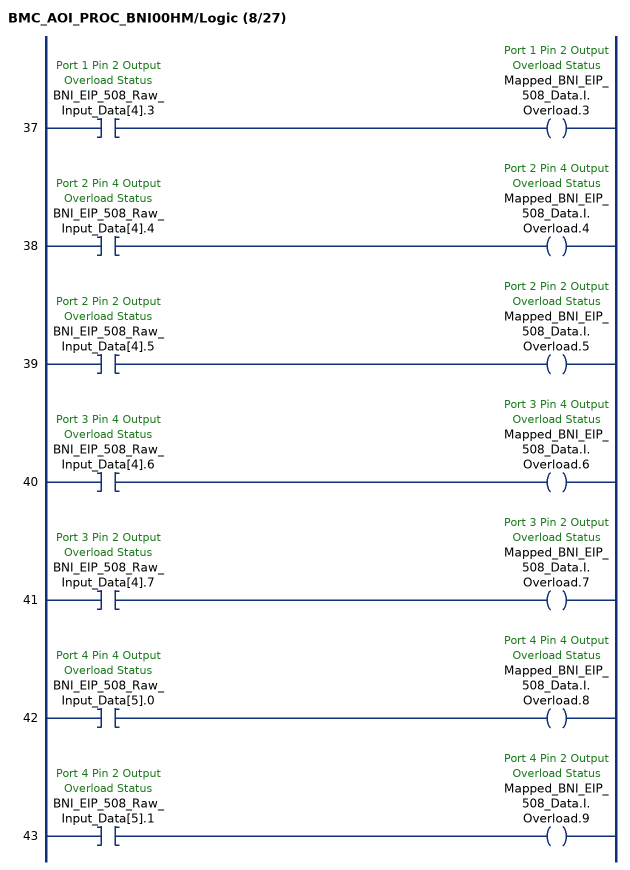
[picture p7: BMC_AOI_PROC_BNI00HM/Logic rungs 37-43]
   37: XIC(BNI_EIP_508_Raw_Input_Data[4].3)OTE(Mapped_BNI_EIP_508_Data.I.Overload.3);
   38: XIC(BNI_EIP_508_Raw_Input_Data[4].4)OTE(Mapped_BNI_EIP_508_Data.I.Overload.4);
   39: XIC(BNI_EIP_508_Raw_Input_Data[4].5)OTE(Mapped_BNI_EIP_508_Data.I.Overload.5);
   40: XIC(BNI_EIP_508_Raw_Input_Data[4].6)OTE(Mapped_BNI_EIP_508_Data.I.Overload.6);
   41: XIC(BNI_EIP_508_Raw_Input_Data[4].7)OTE(Mapped_BNI_EIP_508_Data.I.Overload.7);
   42: XIC(BNI_EIP_508_Raw_Input_Data[5].0)OTE(Mapped_BNI_EIP_508_Data.I.Overload.8);
   43: XIC(BNI_EIP_508_Raw_Input_Data[5].1)OTE(Mapped_BNI_EIP_508_Data.I.Overload.9);
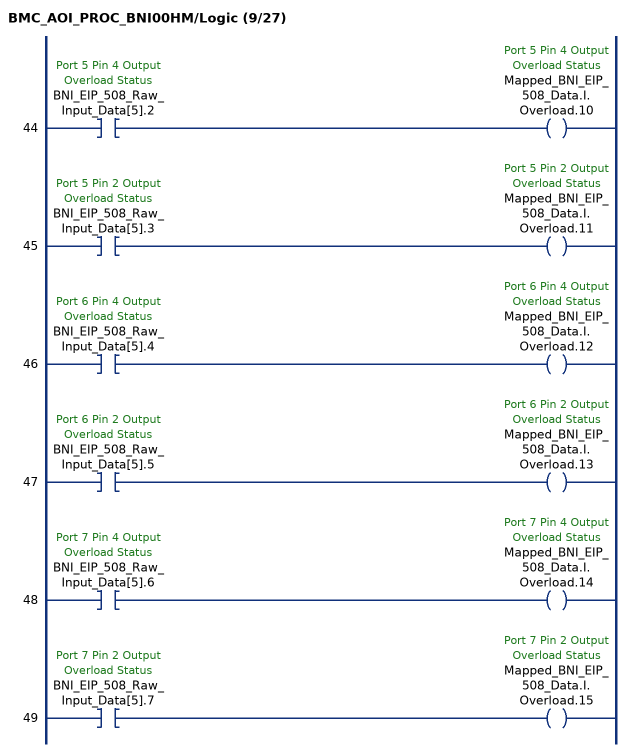
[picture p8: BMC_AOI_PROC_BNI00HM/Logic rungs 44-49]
   44: XIC(BNI_EIP_508_Raw_Input_Data[5].2)OTE(Mapped_BNI_EIP_508_Data.I.Overload.10);
   45: XIC(BNI_EIP_508_Raw_Input_Data[5].3)OTE(Mapped_BNI_EIP_508_Data.I.Overload.11);
   46: XIC(BNI_EIP_508_Raw_Input_Data[5].4)OTE(Mapped_BNI_EIP_508_Data.I.Overload.12);
   47: XIC(BNI_EIP_508_Raw_Input_Data[5].5)OTE(Mapped_BNI_EIP_508_Data.I.Overload.13);
   48: XIC(BNI_EIP_508_Raw_Input_Data[5].6)OTE(Mapped_BNI_EIP_508_Data.I.Overload.14);
   49: XIC(BNI_EIP_508_Raw_Input_Data[5].7)OTE(Mapped_BNI_EIP_508_Data.I.Overload.15);
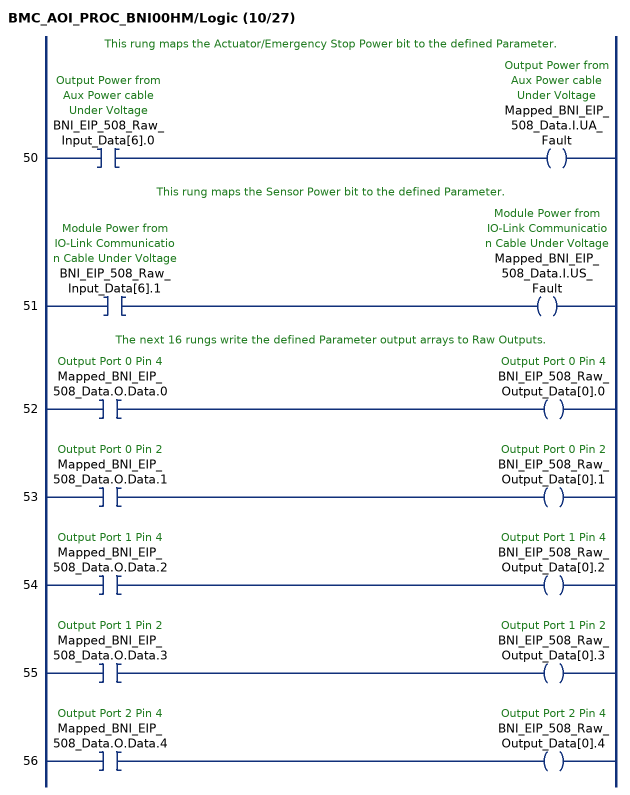
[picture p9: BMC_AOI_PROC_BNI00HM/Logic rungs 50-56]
   // This rung maps the Actuator/Emergency Stop Power bit to the defined Parameter.
   50: XIC(BNI_EIP_508_Raw_Input_Data[6].0)OTE(Mapped_BNI_EIP_508_Data.I.UA_Fault);
   // This rung maps the Sensor Power bit to the defined Parameter.
   51: XIC(BNI_EIP_508_Raw_Input_Data[6].1)OTE(Mapped_BNI_EIP_508_Data.I.US_Fault);
   // The next 16 rungs write the defined Parameter output arrays to Raw Outputs.
   52: XIC(Mapped_BNI_EIP_508_Data.O.Data.0)OTE(BNI_EIP_508_Raw_Output_Data[0].0);
   53: XIC(Mapped_BNI_EIP_508_Data.O.Data.1)OTE(BNI_EIP_508_Raw_Output_Data[0].1);
   54: XIC(Mapped_BNI_EIP_508_Data.O.Data.2)OTE(BNI_EIP_508_Raw_Output_Data[0].2);
   55: XIC(Mapped_BNI_EIP_508_Data.O.Data.3)OTE(BNI_EIP_508_Raw_Output_Data[0].3);
   56: XIC(Mapped_BNI_EIP_508_Data.O.Data.4)OTE(BNI_EIP_508_Raw_Output_Data[0].4);
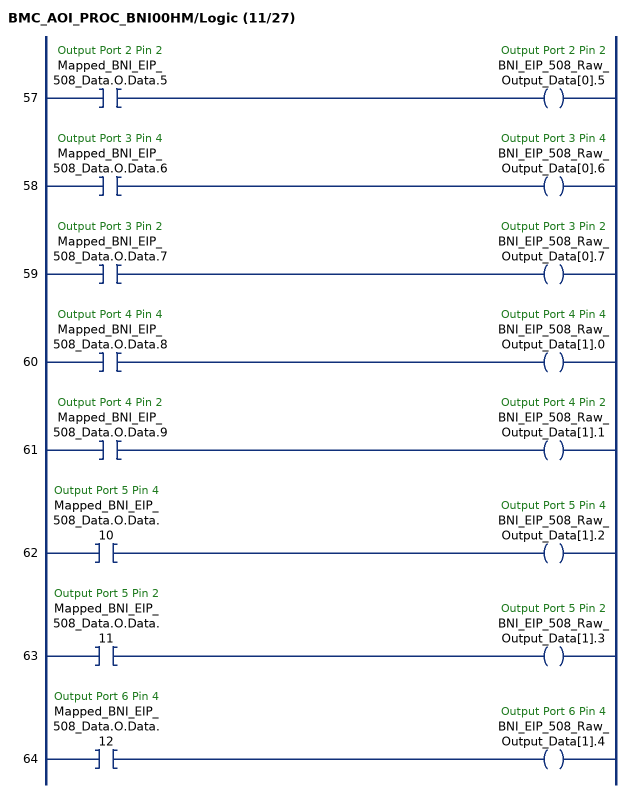
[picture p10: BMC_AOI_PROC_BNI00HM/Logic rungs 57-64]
   57: XIC(Mapped_BNI_EIP_508_Data.O.Data.5)OTE(BNI_EIP_508_Raw_Output_Data[0].5);
   58: XIC(Mapped_BNI_EIP_508_Data.O.Data.6)OTE(BNI_EIP_508_Raw_Output_Data[0].6);
   59: XIC(Mapped_BNI_EIP_508_Data.O.Data.7)OTE(BNI_EIP_508_Raw_Output_Data[0].7);
   60: XIC(Mapped_BNI_EIP_508_Data.O.Data.8)OTE(BNI_EIP_508_Raw_Output_Data[1].0);
   61: XIC(Mapped_BNI_EIP_508_Data.O.Data.9)OTE(BNI_EIP_508_Raw_Output_Data[1].1);
   62: XIC(Mapped_BNI_EIP_508_Data.O.Data.10)OTE(BNI_EIP_508_Raw_Output_Data[1].2);
   63: XIC(Mapped_BNI_EIP_508_Data.O.Data.11)OTE(BNI_EIP_508_Raw_Output_Data[1].3);
   64: XIC(Mapped_BNI_EIP_508_Data.O.Data.12)OTE(BNI_EIP_508_Raw_Output_Data[1].4);
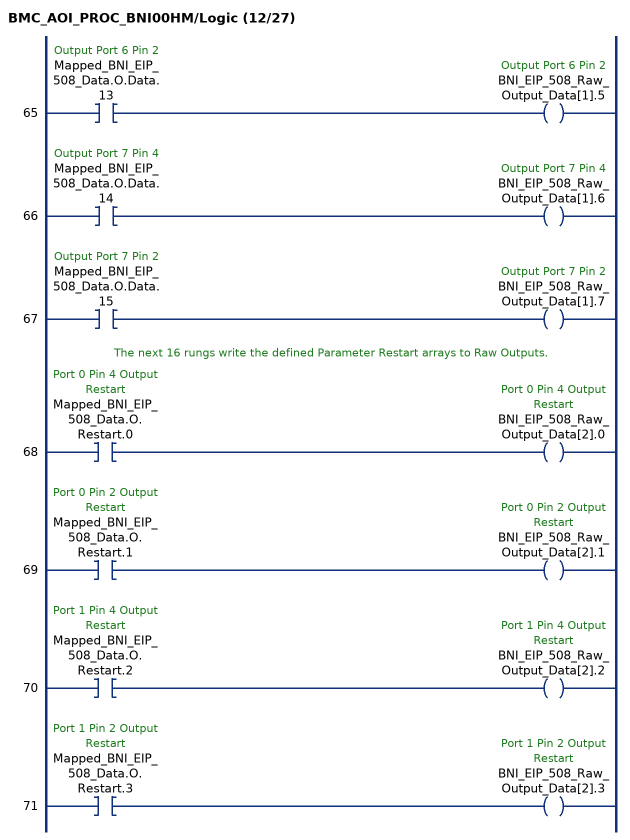
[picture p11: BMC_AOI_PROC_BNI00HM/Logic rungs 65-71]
   65: XIC(Mapped_BNI_EIP_508_Data.O.Data.13)OTE(BNI_EIP_508_Raw_Output_Data[1].5);
   66: XIC(Mapped_BNI_EIP_508_Data.O.Data.14)OTE(BNI_EIP_508_Raw_Output_Data[1].6);
   67: XIC(Mapped_BNI_EIP_508_Data.O.Data.15)OTE(BNI_EIP_508_Raw_Output_Data[1].7);
   // The next 16 rungs write the defined Parameter Restart arrays to Raw Outputs.
   68: XIC(Mapped_BNI_EIP_508_Data.O.Restart.0)OTE(BNI_EIP_508_Raw_Output_Data[2].0);
   69: XIC(Mapped_BNI_EIP_508_Data.O.Restart.1)OTE(BNI_EIP_508_Raw_Output_Data[2].1);
   70: XIC(Mapped_BNI_EIP_508_Data.O.Restart.2)OTE(BNI_EIP_508_Raw_Output_Data[2].2);
   71: XIC(Mapped_BNI_EIP_508_Data.O.Restart.3)OTE(BNI_EIP_508_Raw_Output_Data[2].3);
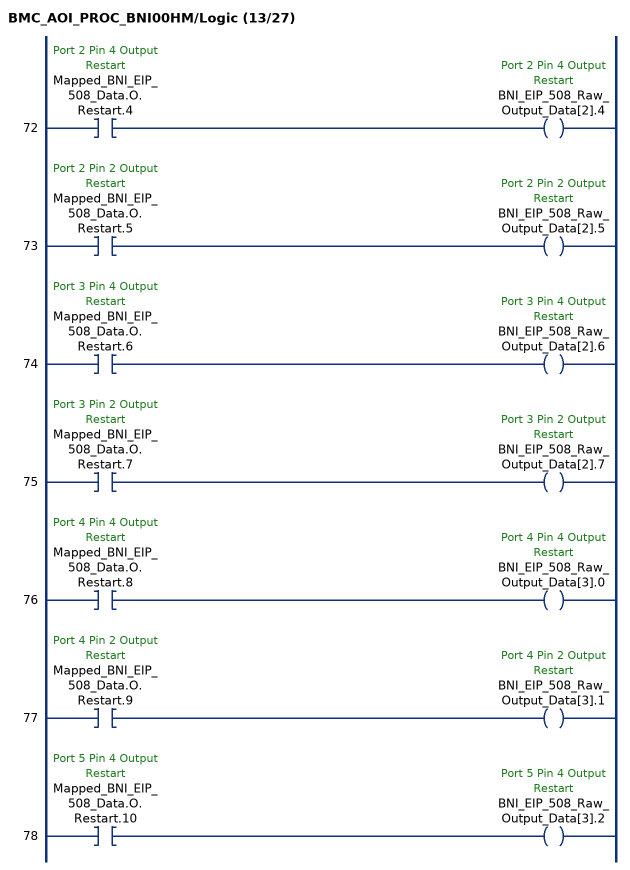
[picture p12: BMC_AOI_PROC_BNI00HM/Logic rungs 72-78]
   72: XIC(Mapped_BNI_EIP_508_Data.O.Restart.4)OTE(BNI_EIP_508_Raw_Output_Data[2].4);
   73: XIC(Mapped_BNI_EIP_508_Data.O.Restart.5)OTE(BNI_EIP_508_Raw_Output_Data[2].5);
   74: XIC(Mapped_BNI_EIP_508_Data.O.Restart.6)OTE(BNI_EIP_508_Raw_Output_Data[2].6);
   75: XIC(Mapped_BNI_EIP_508_Data.O.Restart.7)OTE(BNI_EIP_508_Raw_Output_Data[2].7);
   76: XIC(Mapped_BNI_EIP_508_Data.O.Restart.8)OTE(BNI_EIP_508_Raw_Output_Data[3].0);
   77: XIC(Mapped_BNI_EIP_508_Data.O.Restart.9)OTE(BNI_EIP_508_Raw_Output_Data[3].1);
   78: XIC(Mapped_BNI_EIP_508_Data.O.Restart.10)OTE(BNI_EIP_508_Raw_Output_Data[3].2);
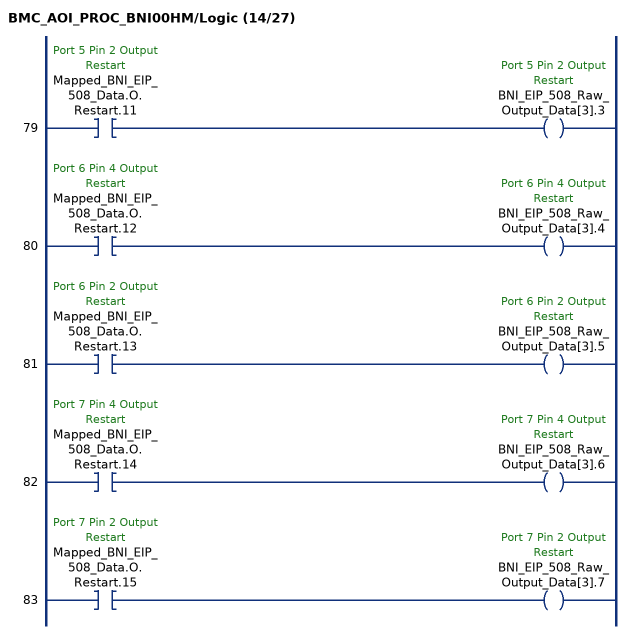
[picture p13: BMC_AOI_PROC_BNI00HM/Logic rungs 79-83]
   79: XIC(Mapped_BNI_EIP_508_Data.O.Restart.11)OTE(BNI_EIP_508_Raw_Output_Data[3].3);
   80: XIC(Mapped_BNI_EIP_508_Data.O.Restart.12)OTE(BNI_EIP_508_Raw_Output_Data[3].4);
   81: XIC(Mapped_BNI_EIP_508_Data.O.Restart.13)OTE(BNI_EIP_508_Raw_Output_Data[3].5);
   82: XIC(Mapped_BNI_EIP_508_Data.O.Restart.14)OTE(BNI_EIP_508_Raw_Output_Data[3].6);
   83: XIC(Mapped_BNI_EIP_508_Data.O.Restart.15)OTE(BNI_EIP_508_Raw_Output_Data[3].7);
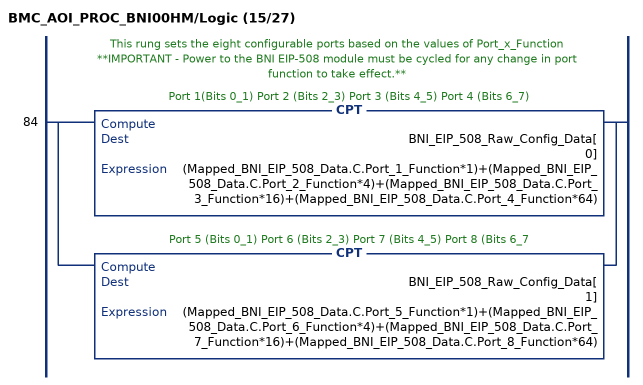
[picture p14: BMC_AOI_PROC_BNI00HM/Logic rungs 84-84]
   // This rung sets the eight configurable ports based on the values of Port_x_Function
   // **IMPORTANT - Power to the BNI EIP-508 module must be cycled for any change in port function to take effect.**
   84: [CPT(BNI_EIP_508_Raw_Config_Data[0],(Mapped_BNI_EIP_508_Data.C.Port_1_Function*1)+(Mapped_BNI_EIP_508_Data.C.Port_2_Function*4)+(Mapped_BNI_EIP_508_Data.C.Port_3_Function*16)+(Mapped_BNI_EIP_508_Data.C.Port_4_Function*64)) ,CPT(BNI_EIP_508_Raw_Config_Data[1],(Mapped_BNI_EIP_508_Data.C.Port_5_Function*1)+(Mapped_BNI_EIP_508_Data.C.Port_6_Function*4)+(Mapped_BNI_EIP_508_Data.C.Port_7_Function*16)+(Mapped_BNI_EIP_508_Data.C.Port_8_Function*64)) ];
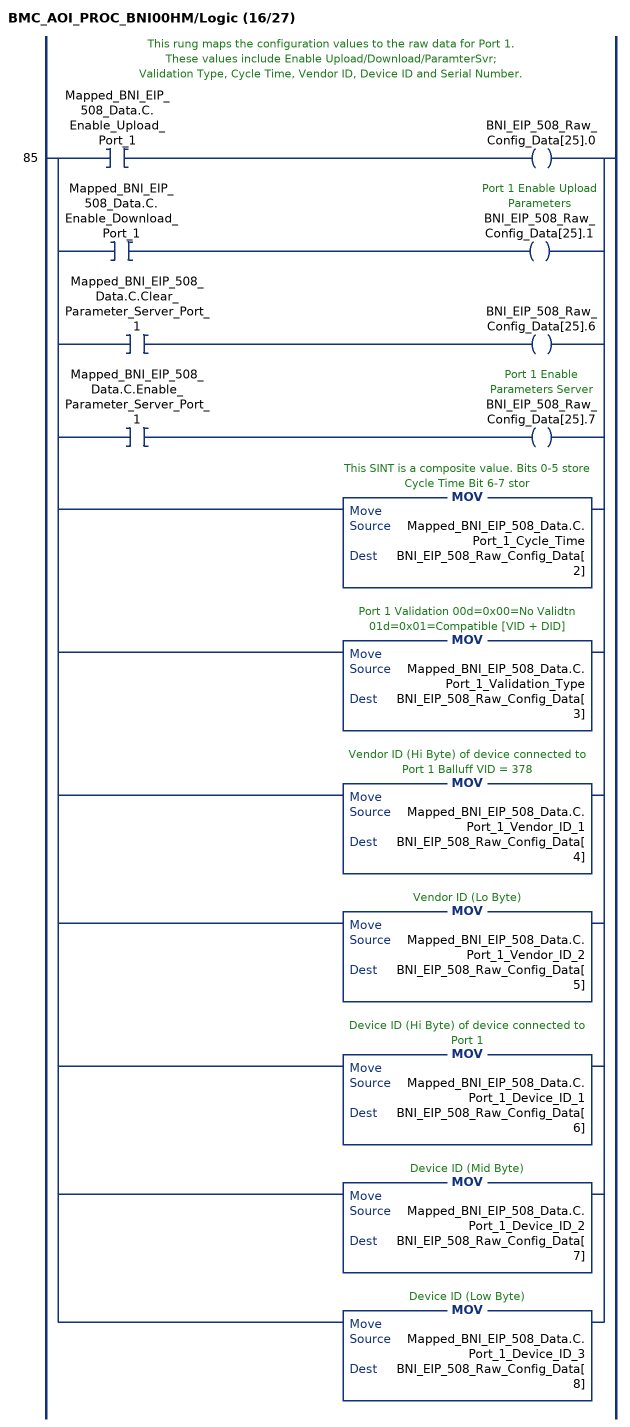
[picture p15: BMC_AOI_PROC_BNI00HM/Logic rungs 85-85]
   // This rung maps the configuration values to the raw data for Port 1.
   // These values include Enable Upload/Download/ParamterSvr;
   // Validation Type, Cycle Time, Vendor ID, Device ID and Serial Number.
   85: [XIC(Mapped_BNI_EIP_508_Data.C.Enable_Upload_Port_1) OTE(BNI_EIP_508_Raw_Config_Data[25].0) ,XIC(Mapped_BNI_EIP_508_Data.C.Enable_Download_Port_1) OTE(BNI_EIP_508_Raw_Config_Data[25].1) ,XIC(Mapped_BNI_EIP_508_Data.C.Clear_Parameter_Server_Port_1) OTE(BNI_EIP_508_Raw_Config_Data[25].6) ,XIC(Mapped_BNI_EIP_508_Data.C.Enable_Parameter_Server_Port_1) OTE(BNI_EIP_508_Raw_Config_Data[25].7) ,MOV(Mapped_BNI_EIP_508_Data.C.Port_1_Cycle_Time,BNI_EIP_508_Raw_Config_Data[2]) ,MOV(Mapped_BNI_EIP_508_Data.C.Port_1_Validation_Type,BNI_EIP_508_Raw_Config_Data[3]) ,MOV(Mapped_BNI_EIP_508_Data.C.Port_1_Vendor_ID_1,BNI_EIP_508_Raw_Config_Data[4]) ,MOV(Mapped_BNI_EIP_508_Data.C.Port_1_Vendor_ID_2,BNI_EIP_508_Raw_Config_Data[5]) ,MOV(Mapped_BNI_EIP_508_Data.C.Port_1_Device_ID_1,BNI_EIP_508_Raw_Config_Data[6]) ,MOV(Mapped_BNI_EIP_508_Data.C.Port_1_Device_ID_2,BNI_EIP_508_Raw_Config_Data[7]) ,MOV(Mapped_BNI_EIP_508_Data.C.Port_1_Device_ID_3,BNI_EIP_508_Raw_Config_Data[8]) ];
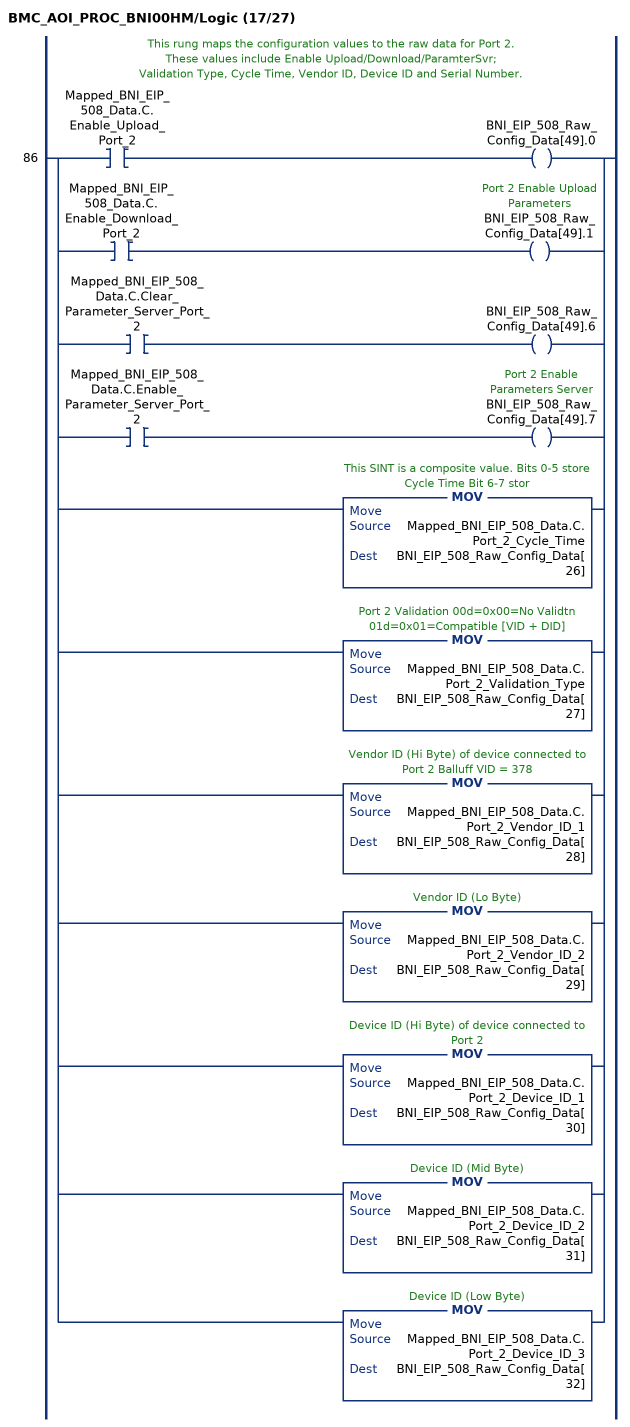
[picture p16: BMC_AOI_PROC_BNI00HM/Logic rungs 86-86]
   // This rung maps the configuration values to the raw data for Port 2.
   // These values include Enable Upload/Download/ParamterSvr;
   // Validation Type, Cycle Time, Vendor ID, Device ID and Serial Number.
   86: [XIC(Mapped_BNI_EIP_508_Data.C.Enable_Upload_Port_2) OTE(BNI_EIP_508_Raw_Config_Data[49].0) ,XIC(Mapped_BNI_EIP_508_Data.C.Enable_Download_Port_2) OTE(BNI_EIP_508_Raw_Config_Data[49].1) ,XIC(Mapped_BNI_EIP_508_Data.C.Clear_Parameter_Server_Port_2) OTE(BNI_EIP_508_Raw_Config_Data[49].6) ,XIC(Mapped_BNI_EIP_508_Data.C.Enable_Parameter_Server_Port_2) OTE(BNI_EIP_508_Raw_Config_Data[49].7) ,MOV(Mapped_BNI_EIP_508_Data.C.Port_2_Cycle_Time,BNI_EIP_508_Raw_Config_Data[26]) ,MOV(Mapped_BNI_EIP_508_Data.C.Port_2_Validation_Type,BNI_EIP_508_Raw_Config_Data[27]) ,MOV(Mapped_BNI_EIP_508_Data.C.Port_2_Vendor_ID_1,BNI_EIP_508_Raw_Config_Data[28]) ,MOV(Mapped_BNI_EIP_508_Data.C.Port_2_Vendor_ID_2,BNI_EIP_508_Raw_Config_Data[29]) ,MOV(Mapped_BNI_EIP_508_Data.C.Port_2_Device_ID_1,BNI_EIP_508_Raw_Config_Data[30]) ,MOV(Mapped_BNI_EIP_508_Data.C.Port_2_Device_ID_2,BNI_EIP_508_Raw_Config_Data[31]) ,MOV(Mapped_BNI_EIP_508_Data.C.Port_2_Device_ID_3,BNI_EIP_508_Raw_Config_Data[32]) ];
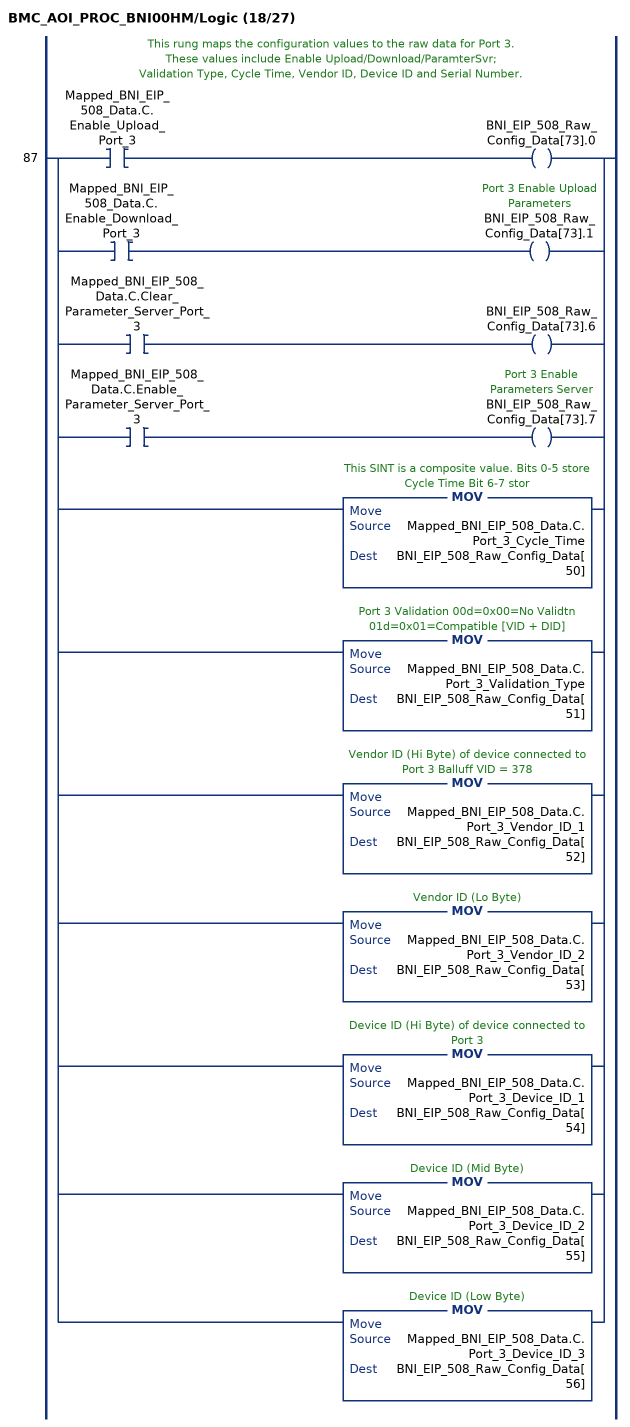
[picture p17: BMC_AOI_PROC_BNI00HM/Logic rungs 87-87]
   // This rung maps the configuration values to the raw data for Port 3.
   // These values include Enable Upload/Download/ParamterSvr;
   // Validation Type, Cycle Time, Vendor ID, Device ID and Serial Number.
   87: [XIC(Mapped_BNI_EIP_508_Data.C.Enable_Upload_Port_3) OTE(BNI_EIP_508_Raw_Config_Data[73].0) ,XIC(Mapped_BNI_EIP_508_Data.C.Enable_Download_Port_3) OTE(BNI_EIP_508_Raw_Config_Data[73].1) ,XIC(Mapped_BNI_EIP_508_Data.C.Clear_Parameter_Server_Port_3) OTE(BNI_EIP_508_Raw_Config_Data[73].6) ,XIC(Mapped_BNI_EIP_508_Data.C.Enable_Parameter_Server_Port_3) OTE(BNI_EIP_508_Raw_Config_Data[73].7) ,MOV(Mapped_BNI_EIP_508_Data.C.Port_3_Cycle_Time,BNI_EIP_508_Raw_Config_Data[50]) ,MOV(Mapped_BNI_EIP_508_Data.C.Port_3_Validation_Type,BNI_EIP_508_Raw_Config_Data[51]) ,MOV(Mapped_BNI_EIP_508_Data.C.Port_3_Vendor_ID_1,BNI_EIP_508_Raw_Config_Data[52]) ,MOV(Mapped_BNI_EIP_508_Data.C.Port_3_Vendor_ID_2,BNI_EIP_508_Raw_Config_Data[53]) ,MOV(Mapped_BNI_EIP_508_Data.C.Port_3_Device_ID_1,BNI_EIP_508_Raw_Config_Data[54]) ,MOV(Mapped_BNI_EIP_508_Data.C.Port_3_Device_ID_2,BNI_EIP_508_Raw_Config_Data[55]) ,MOV(Mapped_BNI_EIP_508_Data.C.Port_3_Device_ID_3,BNI_EIP_508_Raw_Config_Data[56]) ];
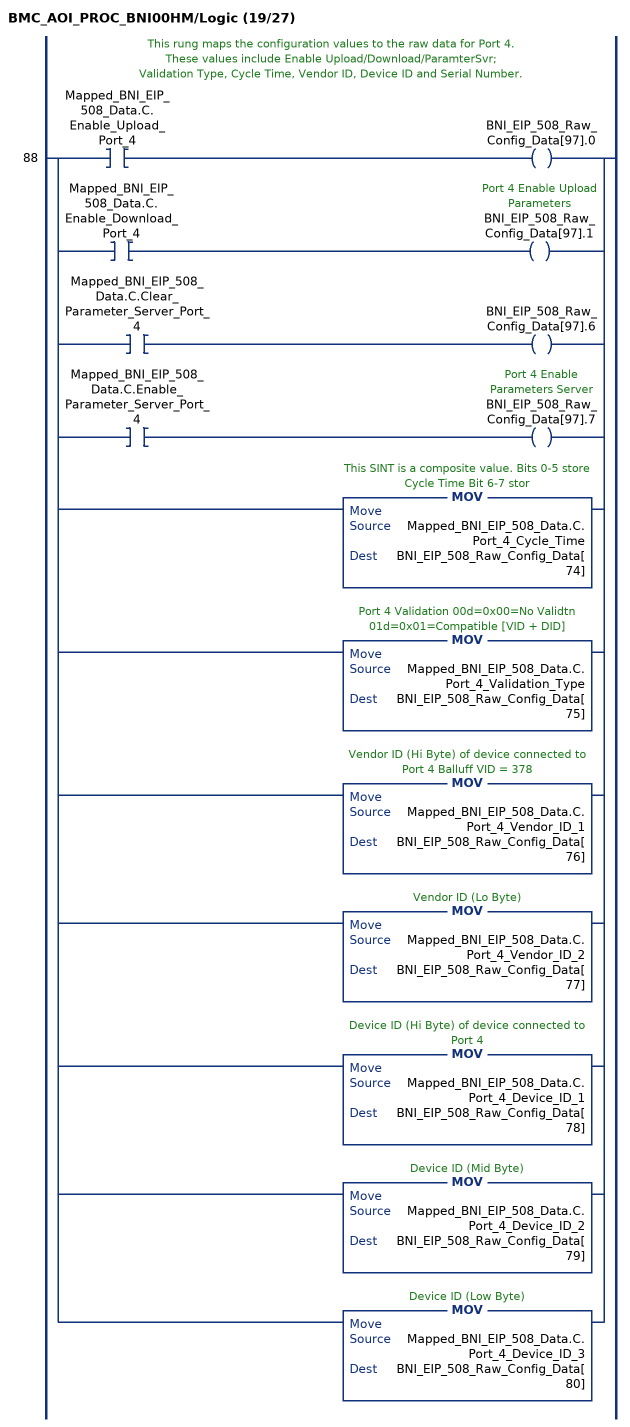
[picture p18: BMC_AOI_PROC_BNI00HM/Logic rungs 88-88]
   // This rung maps the configuration values to the raw data for Port 4.
   // These values include Enable Upload/Download/ParamterSvr;
   // Validation Type, Cycle Time, Vendor ID, Device ID and Serial Number.
   88: [XIC(Mapped_BNI_EIP_508_Data.C.Enable_Upload_Port_4) OTE(BNI_EIP_508_Raw_Config_Data[97].0) ,XIC(Mapped_BNI_EIP_508_Data.C.Enable_Download_Port_4) OTE(BNI_EIP_508_Raw_Config_Data[97].1) ,XIC(Mapped_BNI_EIP_508_Data.C.Clear_Parameter_Server_Port_4) OTE(BNI_EIP_508_Raw_Config_Data[97].6) ,XIC(Mapped_BNI_EIP_508_Data.C.Enable_Parameter_Server_Port_4) OTE(BNI_EIP_508_Raw_Config_Data[97].7) ,MOV(Mapped_BNI_EIP_508_Data.C.Port_4_Cycle_Time,BNI_EIP_508_Raw_Config_Data[74]) ,MOV(Mapped_BNI_EIP_508_Data.C.Port_4_Validation_Type,BNI_EIP_508_Raw_Config_Data[75]) ,MOV(Mapped_BNI_EIP_508_Data.C.Port_4_Vendor_ID_1,BNI_EIP_508_Raw_Config_Data[76]) ,MOV(Mapped_BNI_EIP_508_Data.C.Port_4_Vendor_ID_2,BNI_EIP_508_Raw_Config_Data[77]) ,MOV(Mapped_BNI_EIP_508_Data.C.Port_4_Device_ID_1,BNI_EIP_508_Raw_Config_Data[78]) ,MOV(Mapped_BNI_EIP_508_Data.C.Port_4_Device_ID_2,BNI_EIP_508_Raw_Config_Data[79]) ,MOV(Mapped_BNI_EIP_508_Data.C.Port_4_Device_ID_3,BNI_EIP_508_Raw_Config_Data[80]) ];
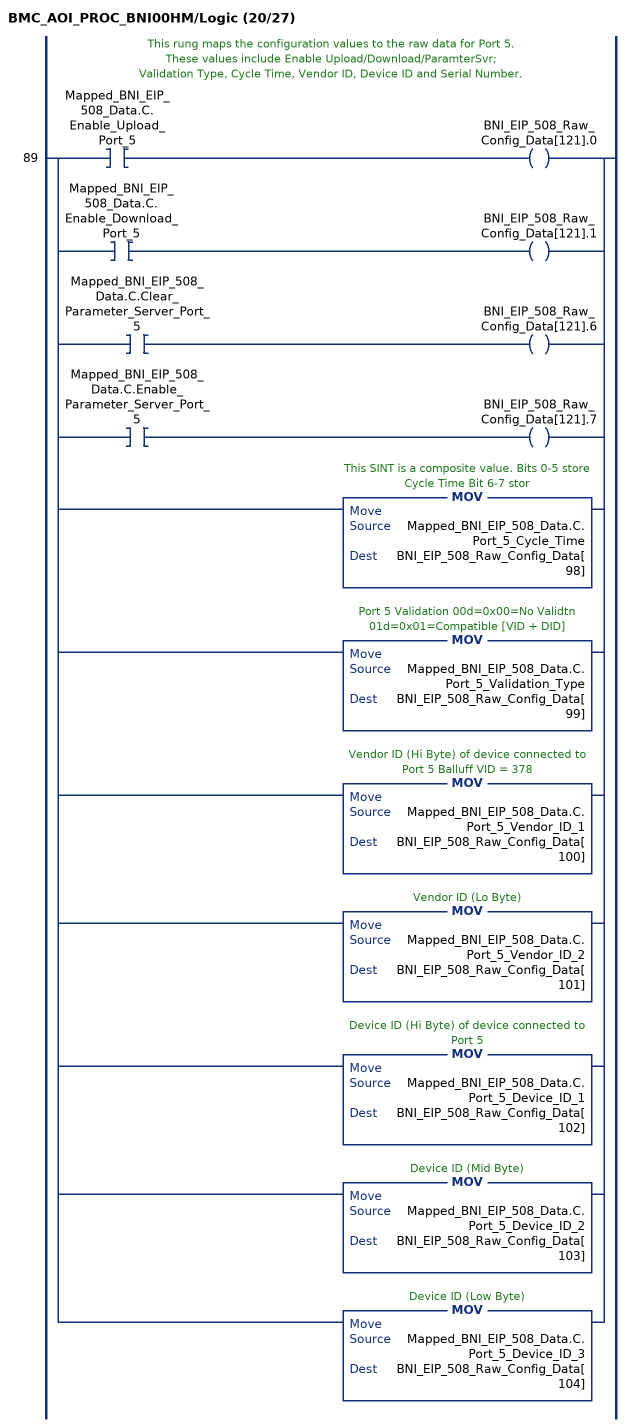
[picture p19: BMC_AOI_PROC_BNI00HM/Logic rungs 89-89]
   // This rung maps the configuration values to the raw data for Port 5.
   // These values include Enable Upload/Download/ParamterSvr;
   // Validation Type, Cycle Time, Vendor ID, Device ID and Serial Number.
   89: [XIC(Mapped_BNI_EIP_508_Data.C.Enable_Upload_Port_5) OTE(BNI_EIP_508_Raw_Config_Data[121].0) ,XIC(Mapped_BNI_EIP_508_Data.C.Enable_Download_Port_5) OTE(BNI_EIP_508_Raw_Config_Data[121].1) ,XIC(Mapped_BNI_EIP_508_Data.C.Clear_Parameter_Server_Port_5) OTE(BNI_EIP_508_Raw_Config_Data[121].6) ,XIC(Mapped_BNI_EIP_508_Data.C.Enable_Parameter_Server_Port_5) OTE(BNI_EIP_508_Raw_Config_Data[121].7) ,MOV(Mapped_BNI_EIP_508_Data.C.Port_5_Cycle_Time,BNI_EIP_508_Raw_Config_Data[98]) ,MOV(Mapped_BNI_EIP_508_Data.C.Port_5_Validation_Type,BNI_EIP_508_Raw_Config_Data[99]) ,MOV(Mapped_BNI_EIP_508_Data.C.Port_5_Vendor_ID_1,BNI_EIP_508_Raw_Config_Data[100]) ,MOV(Mapped_BNI_EIP_508_Data.C.Port_5_Vendor_ID_2,BNI_EIP_508_Raw_Config_Data[101]) ,MOV(Mapped_BNI_EIP_508_Data.C.Port_5_Device_ID_1,BNI_EIP_508_Raw_Config_Data[102]) ,MOV(Mapped_BNI_EIP_508_Data.C.Port_5_Device_ID_2,BNI_EIP_508_Raw_Config_Data[103]) ,MOV(Mapped_BNI_EIP_508_Data.C.Port_5_Device_ID_3,BNI_EIP_508_Raw_Config_Data[104]) ];
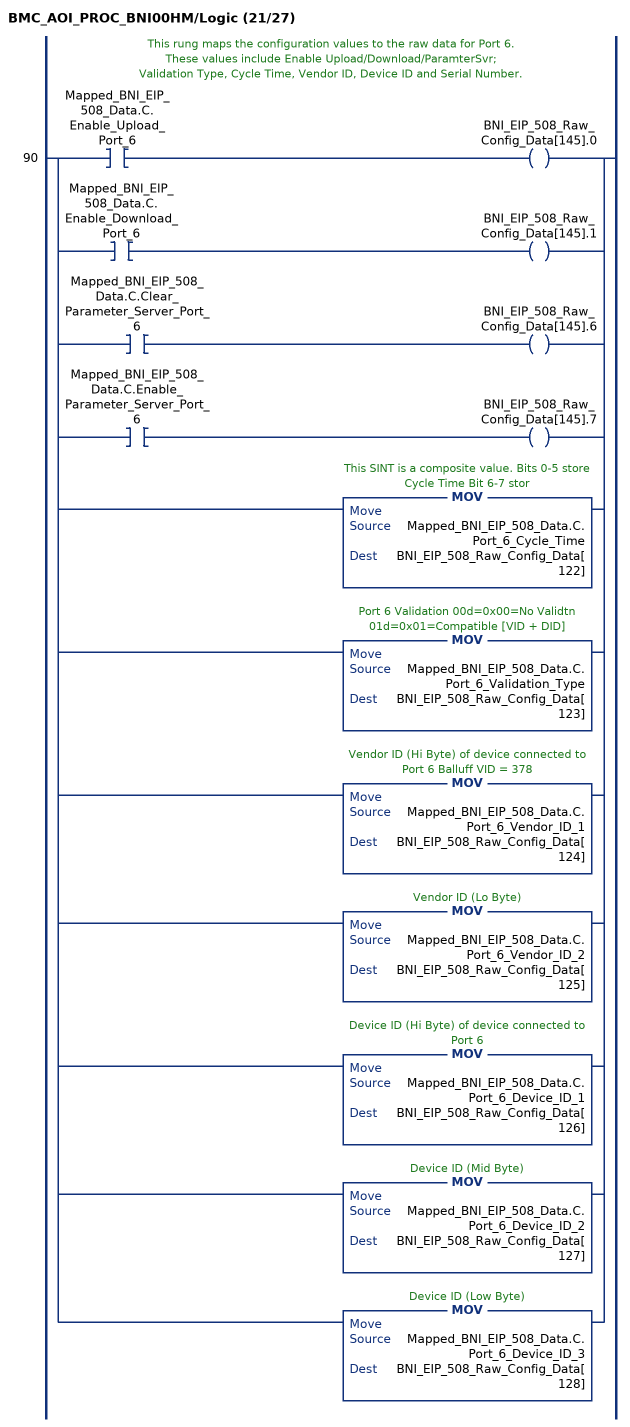
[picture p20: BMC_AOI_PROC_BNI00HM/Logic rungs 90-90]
   // This rung maps the configuration values to the raw data for Port 6.
   // These values include Enable Upload/Download/ParamterSvr;
   // Validation Type, Cycle Time, Vendor ID, Device ID and Serial Number.
   90: [XIC(Mapped_BNI_EIP_508_Data.C.Enable_Upload_Port_6) OTE(BNI_EIP_508_Raw_Config_Data[145].0) ,XIC(Mapped_BNI_EIP_508_Data.C.Enable_Download_Port_6) OTE(BNI_EIP_508_Raw_Config_Data[145].1) ,XIC(Mapped_BNI_EIP_508_Data.C.Clear_Parameter_Server_Port_6) OTE(BNI_EIP_508_Raw_Config_Data[145].6) ,XIC(Mapped_BNI_EIP_508_Data.C.Enable_Parameter_Server_Port_6) OTE(BNI_EIP_508_Raw_Config_Data[145].7) ,MOV(Mapped_BNI_EIP_508_Data.C.Port_6_Cycle_Time,BNI_EIP_508_Raw_Config_Data[122]) ,MOV(Mapped_BNI_EIP_508_Data.C.Port_6_Validation_Type,BNI_EIP_508_Raw_Config_Data[123]) ,MOV(Mapped_BNI_EIP_508_Data.C.Port_6_Vendor_ID_1,BNI_EIP_508_Raw_Config_Data[124]) ,MOV(Mapped_BNI_EIP_508_Data.C.Port_6_Vendor_ID_2,BNI_EIP_508_Raw_Config_Data[125]) ,MOV(Mapped_BNI_EIP_508_Data.C.Port_6_Device_ID_1,BNI_EIP_508_Raw_Config_Data[126]) ,MOV(Mapped_BNI_EIP_508_Data.C.Port_6_Device_ID_2,BNI_EIP_508_Raw_Config_Data[127]) ,MOV(Mapped_BNI_EIP_508_Data.C.Port_6_Device_ID_3,BNI_EIP_508_Raw_Config_Data[128]) ];
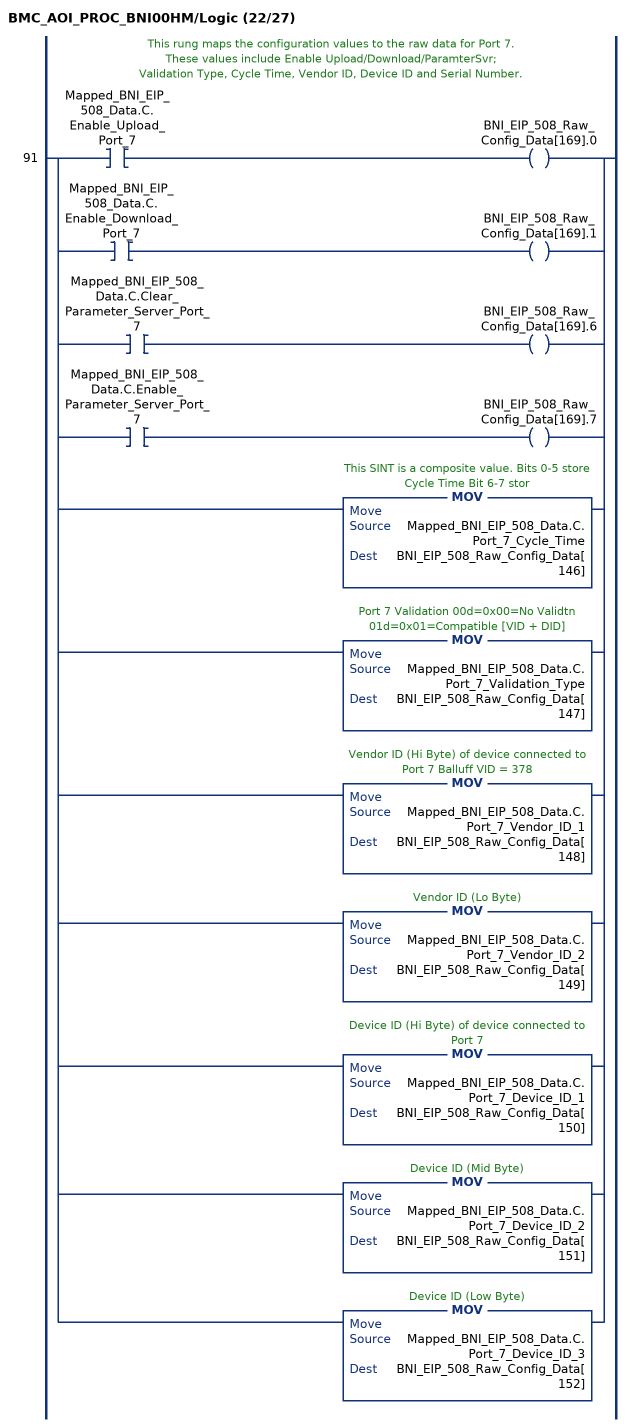
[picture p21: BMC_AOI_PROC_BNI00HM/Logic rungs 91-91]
   // This rung maps the configuration values to the raw data for Port 7.
   // These values include Enable Upload/Download/ParamterSvr;
   // Validation Type, Cycle Time, Vendor ID, Device ID and Serial Number.
   91: [XIC(Mapped_BNI_EIP_508_Data.C.Enable_Upload_Port_7) OTE(BNI_EIP_508_Raw_Config_Data[169].0) ,XIC(Mapped_BNI_EIP_508_Data.C.Enable_Download_Port_7) OTE(BNI_EIP_508_Raw_Config_Data[169].1) ,XIC(Mapped_BNI_EIP_508_Data.C.Clear_Parameter_Server_Port_7) OTE(BNI_EIP_508_Raw_Config_Data[169].6) ,XIC(Mapped_BNI_EIP_508_Data.C.Enable_Parameter_Server_Port_7) OTE(BNI_EIP_508_Raw_Config_Data[169].7) ,MOV(Mapped_BNI_EIP_508_Data.C.Port_7_Cycle_Time,BNI_EIP_508_Raw_Config_Data[146]) ,MOV(Mapped_BNI_EIP_508_Data.C.Port_7_Validation_Type,BNI_EIP_508_Raw_Config_Data[147]) ,MOV(Mapped_BNI_EIP_508_Data.C.Port_7_Vendor_ID_1,BNI_EIP_508_Raw_Config_Data[148]) ,MOV(Mapped_BNI_EIP_508_Data.C.Port_7_Vendor_ID_2,BNI_EIP_508_Raw_Config_Data[149]) ,MOV(Mapped_BNI_EIP_508_Data.C.Port_7_Device_ID_1,BNI_EIP_508_Raw_Config_Data[150]) ,MOV(Mapped_BNI_EIP_508_Data.C.Port_7_Device_ID_2,BNI_EIP_508_Raw_Config_Data[151]) ,MOV(Mapped_BNI_EIP_508_Data.C.Port_7_Device_ID_3,BNI_EIP_508_Raw_Config_Data[152]) ];
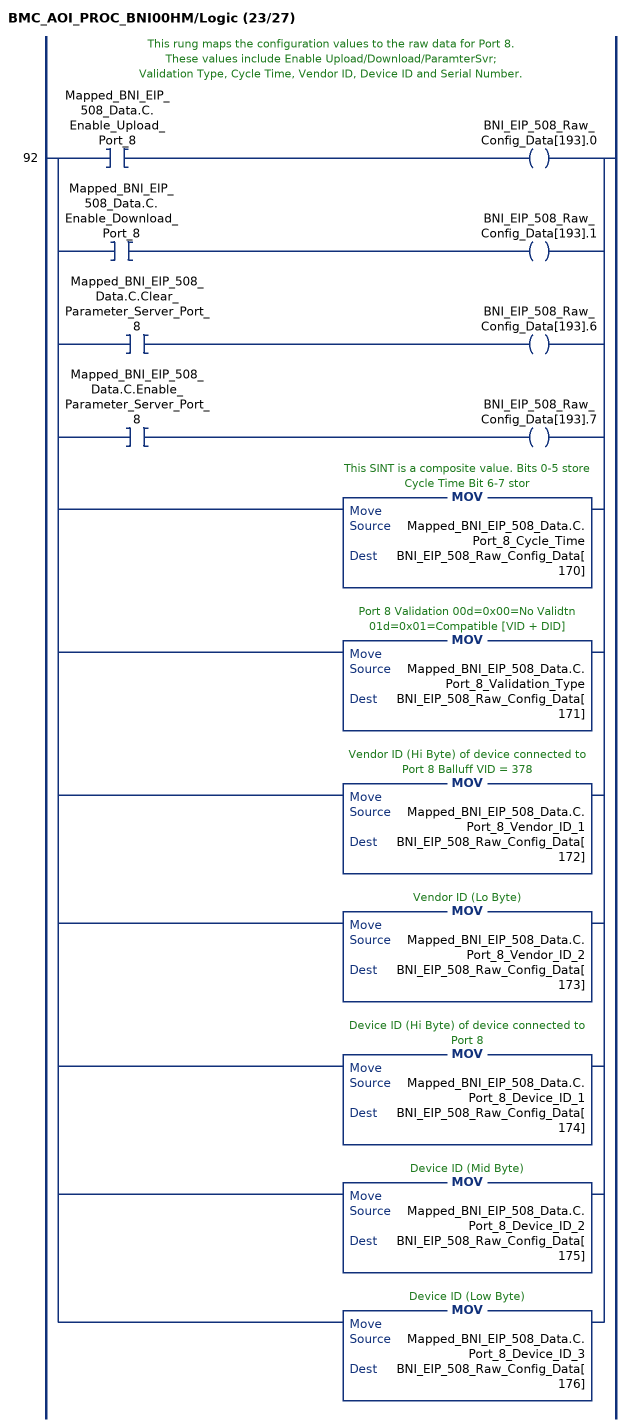
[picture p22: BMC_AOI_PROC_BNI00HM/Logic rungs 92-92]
   // This rung maps the configuration values to the raw data for Port 8.
   // These values include Enable Upload/Download/ParamterSvr;
   // Validation Type, Cycle Time, Vendor ID, Device ID and Serial Number.
   92: [XIC(Mapped_BNI_EIP_508_Data.C.Enable_Upload_Port_8) OTE(BNI_EIP_508_Raw_Config_Data[193].0) ,XIC(Mapped_BNI_EIP_508_Data.C.Enable_Download_Port_8) OTE(BNI_EIP_508_Raw_Config_Data[193].1) ,XIC(Mapped_BNI_EIP_508_Data.C.Clear_Parameter_Server_Port_8) OTE(BNI_EIP_508_Raw_Config_Data[193].6) ,XIC(Mapped_BNI_EIP_508_Data.C.Enable_Parameter_Server_Port_8) OTE(BNI_EIP_508_Raw_Config_Data[193].7) ,MOV(Mapped_BNI_EIP_508_Data.C.Port_8_Cycle_Time,BNI_EIP_508_Raw_Config_Data[170]) ,MOV(Mapped_BNI_EIP_508_Data.C.Port_8_Validation_Type,BNI_EIP_508_Raw_Config_Data[171]) ,MOV(Mapped_BNI_EIP_508_Data.C.Port_8_Vendor_ID_1,BNI_EIP_508_Raw_Config_Data[172]) ,MOV(Mapped_BNI_EIP_508_Data.C.Port_8_Vendor_ID_2,BNI_EIP_508_Raw_Config_Data[173]) ,MOV(Mapped_BNI_EIP_508_Data.C.Port_8_Device_ID_1,BNI_EIP_508_Raw_Config_Data[174]) ,MOV(Mapped_BNI_EIP_508_Data.C.Port_8_Device_ID_2,BNI_EIP_508_Raw_Config_Data[175]) ,MOV(Mapped_BNI_EIP_508_Data.C.Port_8_Device_ID_3,BNI_EIP_508_Raw_Config_Data[176]) ];
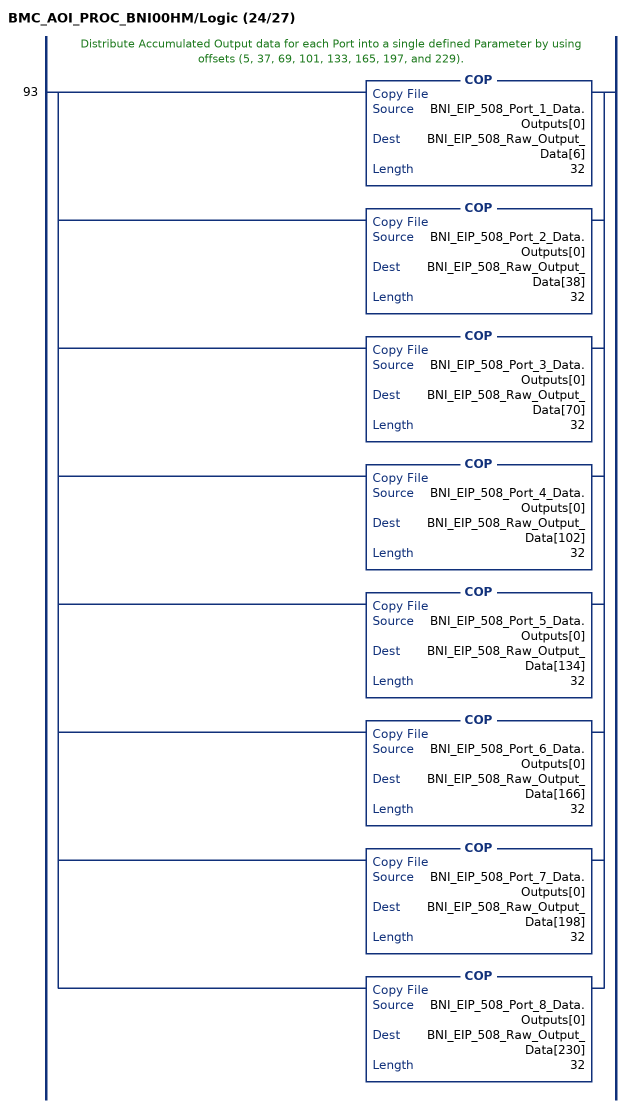
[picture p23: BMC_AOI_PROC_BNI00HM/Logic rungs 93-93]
   // Distribute Accumulated Output data for each Port into a single defined Parameter by using offsets (5, 37, 69, 101, 133, 165, 197, and 229).
   93: [COP(BNI_EIP_508_Port_1_Data.Outputs[0],BNI_EIP_508_Raw_Output_Data[6],32) ,COP(BNI_EIP_508_Port_2_Data.Outputs[0],BNI_EIP_508_Raw_Output_Data[38],32) ,COP(BNI_EIP_508_Port_3_Data.Outputs[0],BNI_EIP_508_Raw_Output_Data[70],32) ,COP(BNI_EIP_508_Port_4_Data.Outputs[0],BNI_EIP_508_Raw_Output_Data[102],32) ,COP(BNI_EIP_508_Port_5_Data.Outputs[0],BNI_EIP_508_Raw_Output_Data[134],32) ,COP(BNI_EIP_508_Port_6_Data.Outputs[0],BNI_EIP_508_Raw_Output_Data[166],32) ,COP(BNI_EIP_508_Port_7_Data.Outputs[0],BNI_EIP_508_Raw_Output_Data[198],32) ,COP(BNI_EIP_508_Port_8_Data.Outputs[0],BNI_EIP_508_Raw_Output_Data[230],32) ];
